DATA_BLOCK "DB_SFB53_FB12"
TITLE =
AUTHOR : SIMATIC
FAMILY : DP
VERSION : 0.1

"WRREC"
BEGIN
   REQ := FALSE;
   ID := DW#16#0;
   INDEX := 0;
   LEN := 0;
   DONE := FALSE;
   BUSY := FALSE;
   ERROR := FALSE;
   STATUS := DW#16#0;
END_DATA_BLOCK

DATA_BLOCK "DB_SFB52_FB10"
TITLE =
AUTHOR : SIMATIC
FAMILY : DP
VERSION : 0.1

"RDREC"
BEGIN
   REQ := FALSE;
   ID := DW#16#0;
   INDEX := 0;
   MLEN := 0;
   VALID := FALSE;
   BUSY := FALSE;
   ERROR := FALSE;
   STATUS := DW#16#0;
   LEN := 0;
END_DATA_BLOCK

DATA_BLOCK "PS_ZYK_DATEN"
TITLE =
VERSION : 0.1
NON_RETAIN


  STRUCT
   Power_Supply : ARRAY  [1 .. 1 ] OF STRUCT
    MESSUNG : STRUCT
     ISTWERT_U : WORD ;
     ISTWERT_I : WORD ;
     ISTWERT_P : WORD ;
    END_STRUCT ;
    PARAMETER : STRUCT
     SCHREIBEN : STRUCT
      SOLLWERT_SPANNUNG : WORD  := W#16#1600;
      SOLLWERT_STROM : WORD  := W#16#A00;
      OPTION_SOLLWERT_LEISTUNG : WORD ;
      OPTION_SOLLWERT_OVP : WORD ;
      OPT_SOLLWERT_WIDERSTAND : WORD ;
     END_STRUCT ;
     LESEN : STRUCT
      STATE : STRUCT
       GERAETEZUSTAND : WORD ;
      END_STRUCT ;
     END_STRUCT ;
    END_STRUCT ;
   END_STRUCT ;
   KONSTANTEN : STRUCT
    LOGISCH_WAHR : BOOL  := TRUE;
    LOGISCH_FALSCH : BOOL ;
   END_STRUCT ;
  END_STRUCT ;
BEGIN
   Power_Supply[1].MESSUNG.ISTWERT_U := W#16#0;
   Power_Supply[1].MESSUNG.ISTWERT_I := W#16#0;
   Power_Supply[1].MESSUNG.ISTWERT_P := W#16#0;
   Power_Supply[1].PARAMETER.SCHREIBEN.SOLLWERT_SPANNUNG := W#16#0;
   Power_Supply[1].PARAMETER.SCHREIBEN.SOLLWERT_STROM := W#16#0;
   Power_Supply[1].PARAMETER.SCHREIBEN.OPTION_SOLLWERT_LEISTUNG := W#16#0;
   Power_Supply[1].PARAMETER.SCHREIBEN.OPTION_SOLLWERT_OVP := W#16#0;
   Power_Supply[1].PARAMETER.SCHREIBEN.OPT_SOLLWERT_WIDERSTAND := W#16#0;
   Power_Supply[1].PARAMETER.LESEN.STATE.GERAETEZUSTAND := W#16#0;
   KONSTANTEN.LOGISCH_WAHR := TRUE;
   KONSTANTEN.LOGISCH_FALSCH := FALSE;
END_DATA_BLOCK

DATA_BLOCK "PS_AZYK_DATEN"
TITLE =
VERSION : 0.1


  STRUCT
   DPV1_Objekte : ARRAY  [1 .. 2 ] OF //vorläufige Platzhaltervariable
   STRUCT
    LESEN : STRUCT
     GERATEDATEN : STRUCT
      GERAETETYP : STRING  [16 ] := 'PSI 9080-100';
      GERAETESERIENNUMMER : STRING  [16 ] := '1026330001';
      GERAETENENNSPANNUNG : REAL  := 8.000000e+001;
      GERAETENENNSTROM : REAL  := 1.000000e+002;
      GERAETEARTIKELNUMMER : STRING  [16 ] := '15200769';
      GERAETEFIRMWARE : STRING  [16 ];
      AKTUELLE_SOLLWERTE : STRUCT
       SPANNUNG : WORD ;
       STROM : WORD ;
       LEISTUNG : WORD ;
      END_STRUCT ;
      GERAETEMELDUNGEN : STRUCT
       KATEGORIE_1 : WORD ;
       CODE_1 : WORD ;
       KATEGORIE_2 : WORD ;
       CODE_2 : WORD ;
       KATEGORIE_3 : WORD ;
       CODE_3 : WORD ;
      END_STRUCT ;
     END_STRUCT ;
    END_STRUCT ;
    SCHREIBEN : STRUCT
     STEUERUNG_GERAET : WORD ;
     SPANNUNGSSOLLWERT : WORD ;
     STROMSOLLWERT : WORD ;
    END_STRUCT ;
   END_STRUCT ;
  END_STRUCT ;
BEGIN
   DPV1_Objekte[1].LESEN.GERATEDATEN.GERAETETYP := 'PSI 9080-100';
   DPV1_Objekte[1].LESEN.GERATEDATEN.GERAETESERIENNUMMER := '';
   DPV1_Objekte[1].LESEN.GERATEDATEN.GERAETENENNSPANNUNG := 0.000000e+000;
   DPV1_Objekte[1].LESEN.GERATEDATEN.GERAETENENNSTROM := 0.000000e+000;
   DPV1_Objekte[1].LESEN.GERATEDATEN.GERAETEARTIKELNUMMER := '';
   DPV1_Objekte[1].LESEN.GERATEDATEN.GERAETEFIRMWARE := '';
   DPV1_Objekte[1].LESEN.GERATEDATEN.AKTUELLE_SOLLWERTE.SPANNUNG := W#16#0;
   DPV1_Objekte[1].LESEN.GERATEDATEN.AKTUELLE_SOLLWERTE.STROM := W#16#0;
   DPV1_Objekte[1].LESEN.GERATEDATEN.AKTUELLE_SOLLWERTE.LEISTUNG := W#16#0;
   DPV1_Objekte[1].LESEN.GERATEDATEN.GERAETEMELDUNGEN.KATEGORIE_1 := W#16#0;
   DPV1_Objekte[1].LESEN.GERATEDATEN.GERAETEMELDUNGEN.CODE_1 := W#16#0;
   DPV1_Objekte[1].LESEN.GERATEDATEN.GERAETEMELDUNGEN.KATEGORIE_2 := W#16#0;
   DPV1_Objekte[1].LESEN.GERATEDATEN.GERAETEMELDUNGEN.CODE_2 := W#16#0;
   DPV1_Objekte[1].LESEN.GERATEDATEN.GERAETEMELDUNGEN.KATEGORIE_3 := W#16#0;
   DPV1_Objekte[1].LESEN.GERATEDATEN.GERAETEMELDUNGEN.CODE_3 := W#16#0;
   DPV1_Objekte[1].SCHREIBEN.STEUERUNG_GERAET := W#16#0;
   DPV1_Objekte[1].SCHREIBEN.SPANNUNGSSOLLWERT := W#16#0;
   DPV1_Objekte[1].SCHREIBEN.STROMSOLLWERT := W#16#0;
   DPV1_Objekte[2].LESEN.GERATEDATEN.GERAETETYP := 'PSI 9080-100';
   DPV1_Objekte[2].LESEN.GERATEDATEN.GERAETESERIENNUMMER := '';
   DPV1_Objekte[2].LESEN.GERATEDATEN.GERAETENENNSPANNUNG := 0.000000e+000;
   DPV1_Objekte[2].LESEN.GERATEDATEN.GERAETENENNSTROM := 0.000000e+000;
   DPV1_Objekte[2].LESEN.GERATEDATEN.GERAETEARTIKELNUMMER := '';
   DPV1_Objekte[2].LESEN.GERATEDATEN.GERAETEFIRMWARE := '';
   DPV1_Objekte[2].LESEN.GERATEDATEN.AKTUELLE_SOLLWERTE.SPANNUNG := W#16#0;
   DPV1_Objekte[2].LESEN.GERATEDATEN.AKTUELLE_SOLLWERTE.STROM := W#16#0;
   DPV1_Objekte[2].LESEN.GERATEDATEN.AKTUELLE_SOLLWERTE.LEISTUNG := W#16#0;
   DPV1_Objekte[2].LESEN.GERATEDATEN.GERAETEMELDUNGEN.KATEGORIE_1 := W#16#0;
   DPV1_Objekte[2].LESEN.GERATEDATEN.GERAETEMELDUNGEN.CODE_1 := W#16#0;
   DPV1_Objekte[2].LESEN.GERATEDATEN.GERAETEMELDUNGEN.KATEGORIE_2 := W#16#0;
   DPV1_Objekte[2].LESEN.GERATEDATEN.GERAETEMELDUNGEN.CODE_2 := W#16#0;
   DPV1_Objekte[2].LESEN.GERATEDATEN.GERAETEMELDUNGEN.KATEGORIE_3 := W#16#0;
   DPV1_Objekte[2].LESEN.GERATEDATEN.GERAETEMELDUNGEN.CODE_3 := W#16#0;
   DPV1_Objekte[2].SCHREIBEN.STEUERUNG_GERAET := W#16#0;
   DPV1_Objekte[2].SCHREIBEN.SPANNUNGSSOLLWERT := W#16#0;
   DPV1_Objekte[2].SCHREIBEN.STROMSOLLWERT := W#16#0;
END_DATA_BLOCK

DATA_BLOCK "WRREC_DB_CONTROLL"
TITLE =
VERSION : 0.1


  STRUCT
   VALID : BOOL ;	//vorläufige Platzhaltervariable
   BUSY : BOOL ;
   ERROR : BOOL ;
   STATUS : DWORD ;
   LAENGE : INT ;
   RECORD : ARRAY  [0 .. 1 ] OF BYTE ;
  END_STRUCT ;
BEGIN
   VALID := FALSE;
   BUSY := FALSE;
   ERROR := FALSE;
   STATUS := DW#16#0;
   LAENGE := 0;
   RECORD[0] := B#16#0;
   RECORD[1] := B#16#0;
END_DATA_BLOCK

DATA_BLOCK "RDREC_DB_DEVICEMESS"
TITLE =
VERSION : 0.1


  STRUCT
   VALID : BOOL ;	//vorläufige Platzhaltervariable
   BUSY : BOOL ;
   ERROR : BOOL ;
   STATUS : DWORD ;
   LAENGE : INT ;
   RECORD : ARRAY  [0 .. 5 ] OF BYTE ;
  END_STRUCT ;
BEGIN
   VALID := FALSE;
   BUSY := FALSE;
   ERROR := FALSE;
   STATUS := DW#16#0;
   LAENGE := 0;
   RECORD[0] := B#16#0;
   RECORD[1] := B#16#0;
   RECORD[2] := B#16#0;
   RECORD[3] := B#16#0;
   RECORD[4] := B#16#0;
   RECORD[5] := B#16#0;
END_DATA_BLOCK

DATA_BLOCK "WRREC_DB_SETVAVOLT"
TITLE =
VERSION : 0.1
NON_RETAIN


  STRUCT
   DONE : BOOL ;	//Datensatz wurde übertragen
   BUSY : BOOL ;	//Schreibvorgang noch nicht beendet (BUSY=1)
   ERROR : BOOL ;	//Schreibvorgang Fehler (ERROR=1)
   STATUS : DWORD ;	//Aufrufkennung / Fehlercode
   RECORD : ARRAY  [0 .. 1 ] OF //Datensatz (zu schreiben)
   BYTE ;
  END_STRUCT ;
BEGIN
   DONE := FALSE;
   BUSY := FALSE;
   ERROR := FALSE;
   STATUS := DW#16#0;
   RECORD[0] := B#16#0;
   RECORD[1] := B#16#0;
END_DATA_BLOCK

DATA_BLOCK "RDREC_DB_ACTSET"
TITLE =
VERSION : 0.1


  STRUCT
   VALID : BOOL ;	//vorläufige Platzhaltervariable
   BUSY : BOOL ;
   ERROR : BOOL ;
   STATUS : DWORD ;
   LAENGE : INT ;
   RECORD : ARRAY  [0 .. 2 ] OF WORD ;
  END_STRUCT ;
BEGIN
   VALID := FALSE;
   BUSY := FALSE;
   ERROR := FALSE;
   STATUS := DW#16#0;
   LAENGE := 0;
   RECORD[0] := W#16#0;
   RECORD[1] := W#16#0;
   RECORD[2] := W#16#0;
END_DATA_BLOCK

DATA_BLOCK "WRREC_DB_SETVACURR"
TITLE =
VERSION : 0.1
NON_RETAIN


  STRUCT
   DONE : BOOL ;	//vorläufige Platzhaltervariable
   BUSY : BOOL ;
   ERROR : BOOL ;
   STATUS : DWORD ;
   RECORD : ARRAY  [0 .. 1 ] OF BYTE ;
  END_STRUCT ;
BEGIN
   DONE := FALSE;
   BUSY := FALSE;
   ERROR := FALSE;
   STATUS := DW#16#0;
   RECORD[0] := B#16#0;
   RECORD[1] := B#16#0;
END_DATA_BLOCK

DATA_BLOCK "RDREC_DB_DEVICETYP"
TITLE =
VERSION : 0.1
NON_RETAIN


  STRUCT
   VALID : BOOL ;	//vorläufige Platzhaltervariable
   BUSY : BOOL ;
   ERROR : BOOL ;
   STATUS : DWORD ;
   LAENGE : INT ;
   RECORD : ARRAY  [0 .. 15 ] OF BYTE ;
  END_STRUCT ;
BEGIN
   VALID := FALSE;
   BUSY := FALSE;
   ERROR := FALSE;
   STATUS := DW#16#0;
   LAENGE := 0;
   RECORD[0] := B#16#0;
   RECORD[1] := B#16#0;
   RECORD[2] := B#16#0;
   RECORD[3] := B#16#0;
   RECORD[4] := B#16#0;
   RECORD[5] := B#16#0;
   RECORD[6] := B#16#0;
   RECORD[7] := B#16#0;
   RECORD[8] := B#16#0;
   RECORD[9] := B#16#0;
   RECORD[10] := B#16#0;
   RECORD[11] := B#16#0;
   RECORD[12] := B#16#0;
   RECORD[13] := B#16#0;
   RECORD[14] := B#16#0;
   RECORD[15] := B#16#0;
END_DATA_BLOCK

DATA_BLOCK "RDREC_DB_DEVARTNO"
TITLE =
VERSION : 0.1
NON_RETAIN


  STRUCT
   VALID : BOOL ;	//vorläufige Platzhaltervariable
   BUSY : BOOL ;
   ERROR : BOOL ;
   STATUS : DWORD ;
   LAENGE : INT ;
   RECORD : ARRAY  [0 .. 15 ] OF BYTE ;
  END_STRUCT ;
BEGIN
   VALID := FALSE;
   BUSY := FALSE;
   ERROR := FALSE;
   STATUS := DW#16#0;
   LAENGE := 0;
   RECORD[0] := B#16#0;
   RECORD[1] := B#16#0;
   RECORD[2] := B#16#0;
   RECORD[3] := B#16#0;
   RECORD[4] := B#16#0;
   RECORD[5] := B#16#0;
   RECORD[6] := B#16#0;
   RECORD[7] := B#16#0;
   RECORD[8] := B#16#0;
   RECORD[9] := B#16#0;
   RECORD[10] := B#16#0;
   RECORD[11] := B#16#0;
   RECORD[12] := B#16#0;
   RECORD[13] := B#16#0;
   RECORD[14] := B#16#0;
   RECORD[15] := B#16#0;
END_DATA_BLOCK

DATA_BLOCK "RDREC_DB_DEVNOMVALUE"
TITLE =
VERSION : 0.1
NON_RETAIN


  STRUCT
   VALID : BOOL ;	//vorläufige Platzhaltervariable
   BUSY : BOOL ;
   ERROR : BOOL ;
   STATUS : DWORD ;
   LAENGE : INT ;
   RECORD : ARRAY  [0 .. 3 ] OF //Nominal Value Voltage
   BYTE ;
  END_STRUCT ;
BEGIN
   VALID := FALSE;
   BUSY := FALSE;
   ERROR := FALSE;
   STATUS := DW#16#0;
   LAENGE := 0;
   RECORD[0] := B#16#0;
   RECORD[1] := B#16#0;
   RECORD[2] := B#16#0;
   RECORD[3] := B#16#0;
END_DATA_BLOCK

DATA_BLOCK "WRREC_DB_SETVAPOW"
TITLE =
VERSION : 0.1


  STRUCT
   DONE : BOOL ;	//vorläufige Platzhaltervariable
   BUSY : BOOL ;
   ERROR : BOOL ;
   STATUS : DWORD ;
   RECORD : ARRAY  [0 .. 1 ] OF BYTE ;
  END_STRUCT ;
BEGIN
   DONE := FALSE;
   BUSY := FALSE;
   ERROR := FALSE;
   STATUS := DW#16#0;
   RECORD[0] := B#16#0;
   RECORD[1] := B#16#0;
END_DATA_BLOCK

DATA_BLOCK "DP_ERROR_DB"
TITLE =
VERSION : 0.1


  STRUCT
   DP_ERROR : BOOL ;	//Slave Fehler
  END_STRUCT ;
BEGIN
   DP_ERROR := FALSE;
END_DATA_BLOCK

FUNCTION "PARA_SPANNUNG_WR" : VOID
TITLE =PARAMETER KONSISTENT SCHREIBEN
VERSION : 0.1


VAR_INPUT
  ADRESSE : INT ;
  DATEN : WORD ;
END_VAR
VAR_TEMP
  _ADRESSE : WORD ;
  _PAFE : INT ;
  _DATEN : WORD ;
END_VAR
BEGIN
NETWORK
TITLE =PARAMETER SPANNUNG SCHREIBEN

      L     #ADRESSE;
      T     #_ADRESSE;

      L     #DATEN;
      T     #_DATEN;

      CALL "DPWR_DAT" (
           LADDR                    := #_ADRESSE,
           RECORD                   := #_DATEN,
           RET_VAL                  := #_PAFE);







END_FUNCTION

FUNCTION "PARA_STROM_WR" : VOID
TITLE =PARAMETER SCHREIBEN
VERSION : 0.1


VAR_INPUT
  ADRESSE : INT ;
  DATEN : WORD ;
END_VAR
VAR_TEMP
  _ADRESSE : WORD ;
  _PAFE : INT ;
  _DATEN : WORD ;
END_VAR
BEGIN
NETWORK
TITLE =PARAMETER STROM SCHREIBEN

      L     #ADRESSE;
      T     #_ADRESSE;

      L     #DATEN;
      T     #_DATEN;

      CALL "DPWR_DAT" (
           LADDR                    := #_ADRESSE,
           RECORD                   := #_DATEN,
           RET_VAL                  := #_PAFE);




END_FUNCTION

FUNCTION "PARA_LEIG_WR" : VOID
TITLE =PARAMETER SCHREIBEN
VERSION : 0.1


VAR_INPUT
  ADRESSE : INT ;
  DATEN : WORD ;
END_VAR
VAR_TEMP
  _ADRESSE : WORD ;
  _PAFE : INT ;
  _DATEN : WORD ;
END_VAR
BEGIN
NETWORK
TITLE =PARAMETER LEISTUNG SCHREIBEN

      L     #ADRESSE;
      T     #_ADRESSE;

      L     #DATEN;
      T     #_DATEN;

      CALL "DPWR_DAT" (
           LADDR                    := #_ADRESSE,
           RECORD                   := P#L 4.0 BYTE 2,
           RET_VAL                  := #_PAFE);

END_FUNCTION

FUNCTION "ISTWERTE_LESEN" : VOID
TITLE =MESSUNG ISTWERTE PS
FAMILY : '        '
NAME : '        '
VERSION : 0.1


VAR_INPUT
  ADRESSE : INT ;
END_VAR
VAR_OUTPUT
  ISTWERT_U : WORD ;
  ISTWERT_I : WORD ;
  ISTWERT_P : WORD ;
END_VAR
VAR_TEMP
  _ADRESSE : WORD ;
  _PAFE : INT ;
  _DATEN : ANY ;
END_VAR
BEGIN
NETWORK
TITLE =ISTWERTE U/I/P LESEN

      L     #ADRESSE;
      T     #_ADRESSE;

      CALL "DPRD_DAT" (
           LADDR                    := #_ADRESSE,
           RET_VAL                  := #_PAFE,
           RECORD                   := P#L 4.0 BYTE 6);//P#DB10.DBX0.0 BYTE 6

      LAR1  P##_DATEN;

      L     LW [AR1,P#0.0];
      T     #ISTWERT_U;

      L     LW [AR1,P#2.0];
      T     #ISTWERT_I;

      L     LW [AR1,P#4.0];
      T     #ISTWERT_P;

END_FUNCTION

FUNCTION "ZUSTAND_LESEN" : VOID
TITLE =GERAETEZUSTAND PS
VERSION : 0.1


VAR_INPUT
  ADRESSE : INT ;
END_VAR
VAR_OUTPUT
  ZUSTAND : WORD ;
END_VAR
VAR_TEMP
  _ADRESSE : WORD ;
  _PAFE : INT ;
  _DATEN : ANY ;
END_VAR
BEGIN
NETWORK
TITLE =GERAETEZUSTAND LESEN

      L     #ADRESSE;
      T     #_ADRESSE;

      CALL "DPRD_DAT" (
           LADDR                    := #_ADRESSE,
           RET_VAL                  := #_PAFE,
           RECORD                   := P#L 4.0 BYTE 2);

      LAR1  P##_DATEN;

      L     LW [AR1,P#0.0];
      T     #ZUSTAND;

END_FUNCTION

FUNCTION "AZYK_WR_SETVALUE" : VOID
TITLE =DPV1 Objekte lesen
VERSION : 0.1


VAR_INPUT
  START : BOOL ;
  ID : DWORD ;
  INDEX : INT ;
  MAX_LAENGE : INT ;
  DBNUMMER : INT ;
END_VAR
VAR_OUTPUT
  DATA_DONE : BOOL ;
  SFB_BUSY : BOOL ;
  SFB_ERROR : BOOL ;
  SFB_STATUS : DWORD ;
END_VAR
VAR_TEMP
  _DBNUMMER : WORD ;
  _MAXLAENGE : INT ;
  _PDATEN : ANY ;
END_VAR
BEGIN
NETWORK
TITLE =

      L     #MAX_LAENGE;
      T     #_MAXLAENGE;

      L     #DBNUMMER;
      T     #_DBNUMMER;

      L     P##_PDATEN;
      LAR1  ;

      L     B#16#10;
      T     B [AR1,P#0.0];

      L     B#16#2;
      T     B [AR1,P#1.0];

      L     #_MAXLAENGE;
      T     W [AR1,P#2.0];

      L     #_DBNUMMER;
      T     W [AR1,P#4.0];

      L     P#DBX 6.0;
      T     D [AR1,P#6.0];

NETWORK
TITLE =

      CALL "WRREC" , "DB_SFB53_FB12" (
           REQ                      := #START,
           ID                       := #ID,
           INDEX                    := #INDEX,
           LEN                      := #_MAXLAENGE,
           DONE                     := #DATA_DONE,
           BUSY                     := #SFB_BUSY,
           ERROR                    := #SFB_ERROR,
           STATUS                   := #SFB_STATUS,
           RECORD                   := #_PDATEN);



END_FUNCTION

FUNCTION "AZYK_WR_CONTROL" : VOID
TITLE =DPV1 Objekte lesen
VERSION : 0.1


VAR_INPUT
  START : BOOL ;
  ID : DWORD ;
  INDEX : INT ;
  MAX_LAENGE : INT ;
  DBNUMMER : INT ;
END_VAR
VAR_OUTPUT
  DATA_DONE : BOOL ;
  SFB_BUSY : BOOL ;
  SFB_ERROR : BOOL ;
  SFB_STATUS : DWORD ;
END_VAR
VAR_TEMP
  _DBNUMMER : WORD ;
  _MAXLAENGE : INT ;
  _PDATEN : ANY ;
END_VAR
BEGIN
NETWORK
TITLE =ANY Zeiger erstellen

      L     #MAX_LAENGE;
      T     #_MAXLAENGE;

      L     #DBNUMMER;
      T     #_DBNUMMER;

      L     P##_PDATEN;
      LAR1  ;

      L     B#16#10;
      T     B [AR1,P#0.0];

      L     B#16#2;
      T     B [AR1,P#1.0];

      L     #_MAXLAENGE;
      T     W [AR1,P#2.0];

      L     #_DBNUMMER;
      T     W [AR1,P#4.0];

      L     P#DBX 8.0;
      T     D [AR1,P#6.0];

NETWORK
TITLE =

      CALL "WRREC" , "DB_SFB53_FB12" (
           REQ                      := #START,
           ID                       := #ID,
           INDEX                    := #INDEX,
           LEN                      := #_MAXLAENGE,
           DONE                     := #DATA_DONE,
           BUSY                     := #SFB_BUSY,
           ERROR                    := #SFB_ERROR,
           STATUS                   := #SFB_STATUS,
           RECORD                   := #_PDATEN);



END_FUNCTION

FUNCTION "AZYK_RD_DEVICEDATA" : VOID
TITLE =
VERSION : 0.1


VAR_INPUT
  START : BOOL ;
  ID : DWORD ;
  INDEX : INT ;
  MAX_LAENGE : INT ;
  DBNUMMER : INT ;
  BITADRESSE : INT ;
  BYTEADRESSE : INT ;
END_VAR
VAR_OUTPUT
  DATA_VALID : BOOL ;
  SFB_BUSY : BOOL ;
  SFB_ERROR : BOOL ;
  SFB_STATUS : DWORD ;
  LAENGE : INT ;
END_VAR
VAR_TEMP
  _DBNUMMER : INT ;
  _MAXLAENGE : INT ;
  _PDATEN : ANY ;
  _BITADRESSE : INT ;
  _BYTEADRESSE : INT ;
END_VAR
BEGIN
NETWORK
TITLE =

      L     #MAX_LAENGE;
      T     #_MAXLAENGE;

      L     #DBNUMMER;
      T     #_DBNUMMER;

      L     #BITADRESSE;
      T     #_BITADRESSE;

      L     #BYTEADRESSE;
      T     #_BYTEADRESSE;

      L     P##_PDATEN;
      LAR1  ;

      L     B#16#10;
      T     B [AR1,P#0.0];

      L     B#16#2;
      T     B [AR1,P#1.0];

      L     #_MAXLAENGE;
      T     W [AR1,P#2.0];

      L     #_DBNUMMER;
      T     W [AR1,P#4.0];

//L     #_BITADRESSE
//UD    DW#16#7
//L     #_BYTEADRESSE
//SLD   3
//OD
//L     B#16#84
//OD
//T     D [AR1,P#6.0]

      L     P#DBX 8.0;
      T     D [AR1,P#6.0];

      CALL "RDREC" , "DB_SFB52_FB10" (
           REQ                      := #START,
           ID                       := #ID,
           INDEX                    := #INDEX,
           MLEN                     := #_MAXLAENGE,
           VALID                    := #DATA_VALID,
           BUSY                     := #SFB_BUSY,
           ERROR                    := #SFB_ERROR,
           STATUS                   := #SFB_STATUS,
           LEN                      := #LAENGE,
           RECORD                   := #_PDATEN);


END_FUNCTION

FUNCTION "AZYK_RD_DEVICENOMVALUE" : VOID
TITLE =
VERSION : 0.1


VAR_INPUT
  START : BOOL ;
  ID : DWORD ;
  INDEX : INT ;
  MAX_LAENGE : INT ;
  DBNUMMER : INT ;
  BITADRESSE : INT ;
  BYTEADRESSE : INT ;
END_VAR
VAR_OUTPUT
  DATA_VALID : BOOL ;
  SFB_BUSY : BOOL ;
  SFB_ERROR : BOOL ;
  SFB_STATUS : DWORD ;
  LAENGE : INT ;
END_VAR
VAR_TEMP
  _DBNUMMER : INT ;
  _MAXLAENGE : INT ;
  _PDATEN : ANY ;
  _BITADRESSE : INT ;
  _BYTEADRESSE : INT ;
END_VAR
BEGIN
NETWORK
TITLE =

      L     #MAX_LAENGE;
      T     #_MAXLAENGE;

      L     #DBNUMMER;
      T     #_DBNUMMER;

      L     #BITADRESSE;
      T     #_BITADRESSE;

      L     #BYTEADRESSE;
      T     #_BYTEADRESSE;

      L     P##_PDATEN;
      LAR1  ;

      L     B#16#10;
      T     B [AR1,P#0.0];

      L     B#16#2;
      T     B [AR1,P#1.0];

      L     #_MAXLAENGE;
      T     W [AR1,P#2.0];

      L     #_DBNUMMER;
      T     W [AR1,P#4.0];

//L     #_BITADRESSE
//UD    DW#16#7
//L     #_BYTEADRESSE
//SLD   3
//OD
//L     B#16#84
//OD
//T     D [AR1,P#6.0]

      L     P#DBX 8.0;
      T     D [AR1,P#6.0];

      CALL "RDREC" , "DB_SFB52_FB10" (
           REQ                      := #START,
           ID                       := #ID,
           INDEX                    := #INDEX,
           MLEN                     := #_MAXLAENGE,
           VALID                    := #DATA_VALID,
           BUSY                     := #SFB_BUSY,
           ERROR                    := #SFB_ERROR,
           STATUS                   := #SFB_STATUS,
           LEN                      := #LAENGE,
           RECORD                   := #_PDATEN);


END_FUNCTION

FUNCTION "AZYK_RD_DATABYTE" : VOID
TITLE =
VERSION : 0.1


VAR_INPUT
  START : BOOL ;
  ID : DWORD ;
  INDEX : INT ;
  MAX_LAENGE : INT ;
  DBNUMMER : INT ;
END_VAR
VAR_OUTPUT
  DATA_VALID : BOOL ;
  SFB_BUSY : BOOL ;
  SFB_ERROR : BOOL ;
  SFB_STATUS : DWORD ;
  LAENGE : INT ;
END_VAR
VAR_TEMP
  _DBNUMMER : INT ;
  _MAXLAENGE : INT ;
  _PDATEN : ANY ;
END_VAR
BEGIN
NETWORK
TITLE =

      L     #MAX_LAENGE;
      T     #_MAXLAENGE;

      L     #DBNUMMER;
      T     #_DBNUMMER;

      L     P##_PDATEN;
      LAR1  ;

      L     B#16#10;
      T     B [AR1,P#0.0];

      L     B#16#2;
      T     B [AR1,P#1.0];

      L     #_MAXLAENGE;
      T     W [AR1,P#2.0];

      L     #_DBNUMMER;
      T     W [AR1,P#4.0];

      L     P#DBX 8.0;
      T     D [AR1,P#6.0];

      CALL "RDREC" , "DB_SFB52_FB10" (
           REQ                      := #START,
           ID                       := #ID,
           INDEX                    := #INDEX,
           MLEN                     := #_MAXLAENGE,
           VALID                    := #DATA_VALID,
           BUSY                     := #SFB_BUSY,
           ERROR                    := #SFB_ERROR,
           STATUS                   := #SFB_STATUS,
           LEN                      := #LAENGE,
           RECORD                   := #_PDATEN);


END_FUNCTION

FUNCTION_BLOCK "PS_ZYKLISCH_DB10"
TITLE =Zyklische Datenverkehr
VERSION : 0.1

BEGIN
NETWORK
TITLE =Messung Istwerte


      CALL "ISTWERTE_LESEN" (
           ADRESSE                  := 256,
           ISTWERT_U                := "PS_ZYK_DATEN".Power_Supply[1].MESSUNG.ISTWERT_U,
           ISTWERT_I                := "PS_ZYK_DATEN".Power_Supply[1].MESSUNG.ISTWERT_I,
           ISTWERT_P                := "PS_ZYK_DATEN".Power_Supply[1].MESSUNG.ISTWERT_P);

NETWORK
TITLE =Geratezustand ermitteln

      CALL "ZUSTAND_LESEN" (
           ADRESSE                  := 262,
           ZUSTAND                  := "PS_ZYK_DATEN".Power_Supply[1].PARAMETER.LESEN.STATE.GERAETEZUSTAND);


END_FUNCTION_BLOCK

FUNCTION "FC10_COPY" : VOID
TITLE =
VERSION : 0.1


VAR_TEMP
  Quelle : ANY ;
  Ziel : ANY ;
END_VAR
BEGIN
NETWORK
TITLE =

      LAR1  P##Quelle;

      L     B#16#10;
      T     LB [AR1,P#0.0];

      L     B#16#2;
      T     LB [AR1,P#1.0];

      L     10;
      T     LW [AR1,P#2.0];

      L     22;
      T     LW [AR1,P#4.0];
      L     P#DBX 11.0;
      T     LD [AR1,P#6.0];

      LAR1  P##Ziel;

      L     B#16#10;
      T     LB [AR1,P#0.0];

      L     B#16#2;
      T     LB [AR1,P#1.0];

      L     10;
      T     LW [AR1,P#2.0];

      L     33;
      T     LW [AR1,P#4.0];
      L     P#DBX 202.0;
      T     LD [AR1,P#6.0];

      CALL "BLKMOV" (
           SRCBLK                   := #Quelle,
           RET_VAL                  := MW    12,
           DSTBLK                   := #Ziel);

END_FUNCTION

FUNCTION_BLOCK "PS_ZYKL_SETVALUE"
TITLE =
VERSION : 0.1

BEGIN
NETWORK
TITLE =Parameter Spannung schreiben


      CALL "PARA_SPANNUNG_WR" (
           ADRESSE                  := 272,
           DATEN                    := "PS_ZYK_DATEN".Power_Supply[1].PARAMETER.SCHREIBEN.SOLLWERT_SPANNUNG);

NETWORK
TITLE =Parameter Strom schreiben


      CALL "PARA_STROM_WR" (
           ADRESSE                  := 274,
           DATEN                    := "PS_ZYK_DATEN".Power_Supply[1].PARAMETER.SCHREIBEN.SOLLWERT_STROM);

NETWORK
TITLE =Parameter Leistung schreiben


      CALL "PARA_LEIG_WR" (
           ADRESSE                  := 276,
           DATEN                    := "PS_ZYK_DATEN".Power_Supply[1].PARAMETER.SCHREIBEN.OPTION_SOLLWERT_LEISTUNG);

END_FUNCTION_BLOCK

FUNCTION_BLOCK "PS_AZYK_SETVAVOLT_WRRD"
TITLE =DPV1 Objekt(e) Sollwert setzen und Aktuelle Sollwerte auslesen
VERSION : 0.1


VAR_OUTPUT
  SFBError : BYTE ;
  SFBStatusOut : DWORD ;
END_VAR
VAR_IN_OUT
  FunctionActivate : BOOL ;	//Anstoßen der Funktion
  FunctionBusy : BOOL ;	//Busybit: Solange TRUE, bis Funktion beendet ist oder TimeOut anspricht
  FunctionDone : BOOL ;	//Zeigt an, daß die Funktion beendet ist (mit oder ohne Fehler)
END_VAR
VAR
  FunctionStaticBusy : BOOL ;	//Speicherbit fuer BusyFlag
  FunctionDPV1WriteDone : BOOL ;
  TimeOutCounter : WORD ;
  SFCRequestLength : INT ;
  FunctionFlag : BOOL ;
END_VAR
VAR_TEMP
  _STATICBusy : BOOL ;
  _SFBError : BOOL ;
  _SFBBusy : BOOL ;
  _SFBDone : BOOL ;
  _SFBValid : BOOL ;
  _SFBStatus : DWORD ;
END_VAR
BEGIN
NETWORK
TITLE =FB Evaluierung

      U     #FunctionActivate;
      FP    #FunctionFlag; // wird weder ein DPV1 Dienst angefragt
      O     #FunctionBusy; // ...noch bearbeitet
      SPBN  END; // so wird der Funktionbaustein beendet
      U     #FunctionStaticBusy; // und wenn zuvor einmal geschrieben wurde
      SPBN  NEWR; // dann NEUE DPV1 ANFRAGE (Request) senden
      U     #FunctionDPV1WriteDone; // Wenn beim DPV1 Dienst WRITE Objekt kein Fehler gemeldet wurde
      SPB   READ; // dann DPV1 Dienst READ Objekt
      SPA   WRIT; // wenn keine READ dann Datensatz schreiben
NEWR: NOP   0; // NEUE DPV1 ANFRAGE (Request)
// Initialisierung
      UN    #FunctionStaticBusy;
      S     #FunctionStaticBusy;
      S     #FunctionBusy;
      R     #FunctionDone;
      L     0;
      T     #SFBError; // Systemfunktionsfehler werden zurueckgesetzt
NETWORK
TITLE =Datensatz Sollwert Spannung setzen

WRIT: NOP   0;
      CALL "AZYK_WR_SETVALUE" (
           START                    := TRUE,
           ID                       := DW#16#108,// PEW276
           INDEX                    := 7,
           MAX_LAENGE               := 2,
           DBNUMMER                 := 153,
           DATA_DONE                := #_SFBDone,
           SFB_BUSY                 := #_SFBBusy,
           SFB_ERROR                := #_SFBError,
           SFB_STATUS               := #_SFBStatus);

// Auswertung der Rueckgabewerte
      U     #_SFBBusy; // wenn die Funktion FC_AZYK_SETVALUE nicht beendet ist,
      SPB   ENDB; // dann Funktionsbaustein Ende
      U     #_SFBError; // wenn Funktion FC_AZYK_SETVALUE keinen Fehler meldet
      SPBN  RD_V; // dann LESEN VORBEREITEN
      SET   ; // Funktion FC_AZYK_SETVALUE hat einen Fehler gemeldet
      R     #FunctionBusy;
      R     #FunctionStaticBusy;
      R     #FunctionDPV1WriteDone;
      S     #FunctionDone;
      L     100; // S7 Fehlercode = 100 laden
      T     #SFBError; // Rueckgabe des Fehlercodes
      L     #_SFBStatus; // Funktionsbaustein Status laden
      T     #SFBStatusOut; // Rückgabe des S7 Fehlercodes
      BEA   ; // Funktionsbaustein wird abgebrochen
// Vorbereiten des des DPV1 Lesedienst
RD_V: NOP   0;
      SET   ;
      S     #FunctionDPV1WriteDone; // nach erfolgreichem WRITEREC Flag setzen

NETWORK
TITLE =Datensatz Aktuelle Sollwerte auslesen

READ: NOP   0;
      CALL "AZYK_RD_DATABYTE" (
           START                    := TRUE,
           ID                       := DW#16#108,// PEW 276
           INDEX                    := 9,
           MAX_LAENGE               := 6,// Anzahl Bytes
           DBNUMMER                 := 154,// Datenbausteinnummer
           DATA_VALID               := #_SFBValid,
           SFB_BUSY                 := #_SFBBusy,
           SFB_ERROR                := #_SFBError,
           SFB_STATUS               := #_SFBStatus,
           LAENGE                   := #SFCRequestLength);

// Auswertung der Rueckgabewerte
      U     #_SFBBusy; // wenn die Funktion FC_AZYKRD_CURRSET nicht beendet ist,
      SPB   ENDB; // dann FunctionBusy Flag setzen
      U     #_SFBError; // wenn bei Datensatz schreiben kein Fehler aufgetreten ist
      SPBN  DATA; // dann Datenauswertung
      L     #TimeOutCounter;
      L     1;
      +I    ;
      T     #TimeOutCounter; // TimeOutCounter += 1
      L     #TimeOutCounter; // Wert von TimeOutCunter laden => AKKU1
      L     300; // Wert 300 laden => AKKU1 => TimeOutCounter => AKKU2
      >=I   ; // VKE = 1 bei AKKU2 >= AKKU1
      SPB   TOUT; // Springe bei VKE = 1 nach TOUT
// wenn der Fehler xx80B5xx gemeldet wird, dann liegt bereits ein anderer DPV1 Auftrag vor
      L     #_SFBStatus;
      UD    DW#16#FFFF00;
      L     DW#16#80B500;
      ==D   ;
// O
//L     #_SFCStatus
//UD    DW#16#FFFF00
//L     DW#16#80B200
//==D
      SPBN  ERR;
      NOP   0;
      SPA   ENDB;
// ein Fehler ist aufgetreten
ERR:  SET   ;
      R     #FunctionBusy;
      R     #FunctionStaticBusy;
      R     #FunctionDPV1WriteDone;
      S     #FunctionDone;
      L     100;
      T     #SFBError;
      L     #_SFBStatus;
      T     #SFBStatusOut;
      L     0;
      T     #TimeOutCounter; // Zeitzähler zurueck setzen
      BEA   ;
DATA: NOP   0;
      S     #FunctionDone;
      R     #FunctionBusy;
      R     #FunctionStaticBusy;
      R     #FunctionDPV1WriteDone;
      R     #FunctionActivate;
      L     0;
      T     #TimeOutCounter;
      BEA   ;

//Timeout
TOUT: NOP   0;
      L     2; // Fehlerwert 2
      T     #SFBError;
      L     0;
      T     #TimeOutCounter; // Zeitzaehler zurueck setzen
      SET   ;
      S     #FunctionDone;
      R     #FunctionActivate;
      R     #FunctionBusy;
      R     #_STATICBusy;
      R     #FunctionDPV1WriteDone;
      BEA   ;
NETWORK
TITLE =Funktionsbaustein definiert beenden

ENDB: SET   ;
      S     #FunctionBusy;
END:  NOP   0;

END_FUNCTION_BLOCK

DATA_BLOCK "DB_FB12_AZYK"
TITLE =
VERSION : 0.1

"PS_AZYK_SETVAVOLT_WRRD"
BEGIN
   SFBError := B#16#0;
   SFBStatusOut := DW#16#0;
   FunctionActivate := FALSE;
   FunctionBusy := FALSE;
   FunctionDone := FALSE;
   FunctionStaticBusy := FALSE;
   FunctionDPV1WriteDone := FALSE;
   TimeOutCounter := W#16#0;
   SFCRequestLength := 0;
   FunctionFlag := FALSE;
END_DATA_BLOCK

FUNCTION_BLOCK "PS_AZYK_SETVACURR_WRRD"
TITLE =DPV1 Objekt(e) Sollwert setzen und Aktuelle Sollwerte auslesen
VERSION : 0.1


VAR_OUTPUT
  SFBError : BYTE ;
  SFBStatusOut : DWORD ;
END_VAR
VAR_IN_OUT
  FunctionActivate : BOOL ;
  FunctionBusy : BOOL ;
  FunctionDone : BOOL ;
END_VAR
VAR
  FunctionStaticBusy : BOOL ;	//SPeicherbit fuer BusyFLag
  FunctionDPV1WriteDone : BOOL ;
  TimeOutCounter : WORD ;
  SFBRequestLength : INT ;
  FunctionFlag : BOOL ;
END_VAR
VAR_TEMP
  _STATICBusy : BOOL ;
  _SFBError : BOOL ;
  _SFBBusy : BOOL ;
  _SFBDone : BOOL ;
  _SFBValid : BOOL ;
  _SFBStatus : DWORD ;
END_VAR
BEGIN
NETWORK
TITLE =FB Evaluierung

      U     #FunctionActivate;
      FP    #FunctionFlag; // wird weder ein DPV1 Dienst angefragt
      O     #FunctionBusy; // ...noch bearbeitet
      SPBN  END; // so wird der Funktionbaustein beendet
      U     #FunctionStaticBusy; // und wenn zuvor einmal geschrieben wurde
      SPBN  NEWR; // dann NEUE DPV1 ANFRAGE (Request) senden
      U     #FunctionDPV1WriteDone; // Wenn beim DPV1 Dienst WRITE Objekt kein Fehler gemeldet wurde
      SPB   READ; // dann DPV1 Dienst READ Objekt
      SPA   WRIT; // wenn keine READ dann Datensatz schreiben
NEWR: NOP   0; // NEUE DPV1 ANFRAGE (Request)
// Initialisierung
      UN    #FunctionStaticBusy;
      S     #FunctionStaticBusy;
      S     #FunctionBusy;
      R     #FunctionDone;
      L     0;
      T     #SFBError; // Systemfunktionsfehler werden zurueckgesetzt

NETWORK
TITLE =Datensatz Sollwert Strom setzen

WRIT: NOP   0;
      CALL "AZYK_WR_SETVALUE" (
           START                    := TRUE,
           ID                       := DW#16#108,
           INDEX                    := 8,
           MAX_LAENGE               := 2,// Anzahl Bytes
           DBNUMMER                 := 155,// Datenbausteinnummer
           DATA_DONE                := #_SFBDone,
           SFB_BUSY                 := #_SFBBusy,
           SFB_ERROR                := #_SFBError,
           SFB_STATUS               := #_SFBStatus);

// Auswertung der Rueckgabewerte
      U     #_SFBBusy; // wenn die Funktion FC_AZYK_SETVALUE nicht beendet ist,
      SPB   ENDB; // dann Funktionsbaustein Ende
      U     #_SFBError; // wenn Funktion FC_AZYK_SETVALUE keinen Fehler meldet
      SPBN  RD_V; // dann LESEN VORBEREITEN
      SET   ; // Funktion FC_AZYK_SETVALUE hat einen Fehler gemeldet
      R     #FunctionBusy;
      R     #FunctionStaticBusy;
      R     #FunctionDPV1WriteDone;
      S     #FunctionDone;
      L     100; // S7 Fehlercode = 100 laden
      T     #SFBError; // Rueckgabe des Fehlercodes
      L     #_SFBStatus; // Funktionsbaustein Status laden
      T     #SFBStatusOut; // Rückgabe des S7 Fehlercodes
      BEA   ; // Funktionsbaustein wird abgebrochen
// Vorbereiten des DPV1 Lesedienst
RD_V: NOP   0;
      SET   ;
      S     #FunctionDPV1WriteDone; // nach erfolgreichem WRITEREC Flag setzen

NETWORK
TITLE =Datensatz Aktuelle Sollwerte auslesen

READ: NOP   0;
      CALL "AZYK_RD_DATABYTE" (
           START                    := TRUE,
           ID                       := DW#16#108,
           INDEX                    := 9,
           MAX_LAENGE               := 6,// Anzahl Bytes
           DBNUMMER                 := 154,// Datenbausteinnummer
           DATA_VALID               := #_SFBValid,
           SFB_BUSY                 := #_SFBBusy,
           SFB_ERROR                := #_SFBError,
           SFB_STATUS               := #_SFBStatus,
           LAENGE                   := #SFBRequestLength);

// Auswertung der Rueckgabewerte
      U     #_SFBBusy; // wenn die Funktion FC_AZYKRD_CURRSET nicht beendet ist,
      SPB   ENDB; // dann FunctionBusy Flag setzen
      U     #_SFBError; // wenn bei Datensatz schreiben kein Fehler aufgetreten ist
      SPBN  DATA; // dann Datenauswertung
      L     #TimeOutCounter;
      L     1;
      +I    ;
      T     #TimeOutCounter; // TimeOutCounter += 1
      L     #TimeOutCounter; // Wert von TimeOutCunter laden => AKKU1
      L     300; // Wert 300 laden => AKKU1 => TimeOutCounter => AKKU2
      >=I   ; // VKE = 1 bei AKKU2 >= AKKU1
      SPB   TOUT; // Springe bei VKE = 1 nach TOUT
// wenn der Fehler xx80B5xx gemeldet wird, dann liegt bereits ein anderer DPV1 Auftrag vor
      L     #_SFBStatus;
      UD    DW#16#FFFF00;
      L     DW#16#80B500;
      ==D   ;
// O
//L     #_SFCStatus
//UD    DW#16#FFFF00
//L     DW#16#80B200
//==D
      SPBN  ERR;
      NOP   0;
      SPA   ENDB;
// ein Fehler ist aufgetreten
ERR:  SET   ;
      R     #FunctionBusy;
      R     #FunctionStaticBusy;
      R     #FunctionDPV1WriteDone;
      S     #FunctionDone;
      L     100;
      T     #SFBError;
      L     #_SFBStatus;
      T     #SFBStatusOut;
      L     0;
      T     #TimeOutCounter; // Zeitzähler zurueck setzen
      BEA   ;
DATA: NOP   0;
      S     #FunctionDone;
      R     #FunctionBusy;
      R     #FunctionStaticBusy;
      R     #FunctionDPV1WriteDone;
      R     #FunctionActivate;
      L     0;
      T     #TimeOutCounter;
      BEA   ;

//Timeout
TOUT: NOP   0;
      L     2; // Fehlerwert 2
      T     #SFBError;
      L     0;
      T     #TimeOutCounter; // Zeitzaehler zurueck setzen
      SET   ;
      S     #FunctionDone;
      R     #FunctionActivate;
      R     #FunctionBusy;
      R     #_STATICBusy;
      R     #FunctionDPV1WriteDone;
      BEA   ;
NETWORK
TITLE =Funktionsbaustein definiert beenden

ENDB: SET   ;
      S     #FunctionBusy;
END:  NOP   0;

END_FUNCTION_BLOCK

DATA_BLOCK "DB_FB13_AZYK"
TITLE =
VERSION : 0.0

"PS_AZYK_SETVACURR_WRRD"
BEGIN
   SFBError := B#16#0;
   SFBStatusOut := DW#16#0;
   FunctionActivate := FALSE;
   FunctionBusy := FALSE;
   FunctionDone := FALSE;
   FunctionStaticBusy := FALSE;
   FunctionDPV1WriteDone := FALSE;
   TimeOutCounter := W#16#0;
   SFBRequestLength := 0;
   FunctionFlag := FALSE;
END_DATA_BLOCK

FUNCTION_BLOCK "PS_AZYK_CONTROLL_WRRD"
TITLE =DPV1 Objekt Geraet Steuerung
VERSION : 0.1


VAR_INPUT
  DBNummer_STEUERN : INT ;
  Datensatznr_STEUERN : INT ;
  DBNummer_MELDUNGEN : INT ;
  Datensatznr_MELDUNGEN : INT ;
END_VAR
VAR_OUTPUT
  SFBError : BYTE ;
  SFBStatusOut : DWORD ;
END_VAR
VAR_IN_OUT
  FunctionActivate : BOOL ;
  FunctionBusy : BOOL ;
  FunctionDone : BOOL ;
END_VAR
VAR
  FunctionStaticBusy : BOOL ;	//SPeicherbit fuer BusyFLag
  FunctionDPV1WriteDone : BOOL ;
  TimeOutCounter : WORD ;
  SFBRequestLength : INT ;
  FunctionFlag : BOOL ;
END_VAR
VAR_TEMP
  _STATICBusy : BOOL ;
  _SFBError : BOOL ;
  _SFBBusy : BOOL ;
  _SFBDone : BOOL ;
  _SFBValid : BOOL ;
  _SFBStatus : DWORD ;
END_VAR
BEGIN
NETWORK
TITLE =FB Evaluierung

      U     #FunctionActivate;
      FP    #FunctionFlag; // wird weder ein DPV1 Dienst angefragt
      O     #FunctionBusy; // ...noch bearbeitet
      SPBN  END; // so wird der Funktionbaustein beendet
      U     #FunctionStaticBusy; // und wenn zuvor einmal geschrieben wurde
      SPBN  NEWR; // dann NEUE DPV1 ANFRAGE (Request) senden
      U     #FunctionDPV1WriteDone; // Wenn beim DPV1 Dienst WRITE Objekt kein Fehler gemeldet wurde
      SPB   READ; // dann DPV1 Dienst READ Objekt
      SPA   WRIT; // wenn keine READ dann Datensatz schreiben
NEWR: NOP   0; // NEUE DPV1 ANFRAGE (Request)
// Initialisierung
      UN    #FunctionStaticBusy;
      S     #FunctionStaticBusy;
      S     #FunctionBusy;
      R     #FunctionDone;
      L     0;
      T     #SFBError; // Systemfunktionsfehler werden zurueckgesetzt

NETWORK
TITLE =Datensatz Geraet steuern

WRIT: NOP   0;
      CALL "AZYK_WR_CONTROL" (
           START                    := TRUE,
           ID                       := DW#16#108,
           INDEX                    := #Datensatznr_STEUERN,
           MAX_LAENGE               := 2,
           DBNUMMER                 := #DBNummer_STEUERN,
           DATA_DONE                := #_SFBDone,
           SFB_BUSY                 := #_SFBBusy,
           SFB_ERROR                := #_SFBError,
           SFB_STATUS               := #_SFBStatus);


// Auswertung der Rueckgabewerte
      U     #_SFBBusy; // wenn die Funktion FC_AZYK_SETVALUE nicht beendet ist,
      SPB   ENDB; // dann Funktionsbaustein Ende
      U     #_SFBError; // wenn Funktion FC_AZYK_SETVALUE keinen Fehler meldet
      SPBN  RD_V; // dann LESEN VORBEREITEN
      SET   ; // Funktion FC_AZYK_SETVALUE hat einen Fehler gemeldet
      R     #FunctionBusy;
      R     #FunctionStaticBusy;
      R     #FunctionDPV1WriteDone;
      S     #FunctionDone;
      L     100; // Fehlercode = 100 laden
      T     #SFBError; // Rueckgabe des Fehlercodes
      L     #_SFBStatus; // Funktionsbaustein Status laden
      T     #SFBStatusOut; // Rückgabe des Statuswert
      BEA   ; // Funktionsbaustein wird abgebrochen
// Vorbereiten des des DPV1 Lesedienst
RD_V: NOP   0;
      SET   ;
      S     #FunctionDPV1WriteDone; // nach erfolgreichem WRITEREC Flag setzen

NETWORK
TITLE =Datensatz Geraetemeldungen auslesen

READ: NOP   0;
      CALL "AZYK_RD_DATABYTE" (
           START                    := TRUE,
           ID                       := DW#16#108,
           INDEX                    := #Datensatznr_MELDUNGEN,
           MAX_LAENGE               := 6,// Anzahl in Bytes
           DBNUMMER                 := #DBNummer_MELDUNGEN,// Datenbausteinnummer
           DATA_VALID               := #_SFBValid,
           SFB_BUSY                 := #_SFBBusy,
           SFB_ERROR                := #_SFBError,
           SFB_STATUS               := #_SFBStatus,
           LAENGE                   := #SFBRequestLength);

// Auswertung der Rueckgabewerte
      U     #_SFBBusy; // wenn die Funktion FC_AZYKRD_CURRSET nicht beendet ist,
      SPB   ENDB; // dann FunctionBusy Flag setzen
      U     #_SFBError; // wenn bei Datensatz schreiben kein Fehler aufgetreten ist
      SPBN  DATA; // dann Datenauswertung
      L     #TimeOutCounter;
      L     1;
      +I    ;
      T     #TimeOutCounter; // TimeOutCounter += 1
      L     #TimeOutCounter; // Wert von TimeOutCunter laden => AKKU1
      L     300; // Wert 300 laden => AKKU1 => TimeOutCounter => AKKU2
      >=I   ; // VKE = 1 bei AKKU2 >= AKKU1
      SPB   TOUT; // Springe bei VKE = 1 nach TOUT
// wenn der Fehler xx80B5xx gemeldet wird, dann liegt bereits ein anderer DPV1 Auftrag vor
      L     #_SFBStatus;
      UD    DW#16#FFFF00;
      L     DW#16#80B500;
      ==D   ;
      O     ;
// wenn der Fehler xx80B2xx gemeldet wird, ist die vorliegende Projektierung der Steckplatzdefinition fehlerhaft
//      L     #_SFBStatus
//      UD    DW#16#FFFF00
//      L     DW#16#80B200
//      ==D
      SPBN  ERR;
      NOP   0;
      SPA   ENDB;
// ein Fehler ist aufgetreten
ERR:  SET   ;
      R     #FunctionBusy;
      R     #FunctionStaticBusy;
      R     #FunctionDPV1WriteDone;
      S     #FunctionDone;
      L     100;
      T     #SFBError;
      L     #_SFBStatus;
      T     #SFBStatusOut;
      L     0;
      T     #TimeOutCounter; // Zeitzähler zurueck setzen
      BEA   ;
DATA: NOP   0;
      S     #FunctionDone;
      R     #FunctionBusy;
      R     #FunctionStaticBusy;
      R     #FunctionDPV1WriteDone;
      R     #FunctionActivate;
      L     0;
      T     #TimeOutCounter; // Zeitzähler zurück setzen
      BEA   ;

//Timeout
TOUT: NOP   0;
      L     2; // Fehlerwert 2
      T     #SFBError;
      L     0;
      T     #TimeOutCounter; // Zeitzaehler zurueck setzen
      SET   ;
      S     #FunctionDone;
      R     #FunctionActivate;
      R     #FunctionBusy;
      R     #_STATICBusy;
      R     #FunctionDPV1WriteDone;
      BEA   ;
NETWORK
TITLE =Funktionsbaustein definiert beenden

ENDB: SET   ;
      S     #FunctionBusy;
END:  NOP   0;

END_FUNCTION_BLOCK

DATA_BLOCK "DB_FB14_AZYK"
TITLE =
VERSION : 0.0

"PS_AZYK_CONTROLL_WRRD"
BEGIN
   DBNummer_STEUERN := 0;
   Datensatznr_STEUERN := 0;
   DBNummer_MELDUNGEN := 0;
   Datensatznr_MELDUNGEN := 0;
   SFBError := B#16#0;
   SFBStatusOut := DW#16#0;
   FunctionActivate := FALSE;
   FunctionBusy := FALSE;
   FunctionDone := FALSE;
   FunctionStaticBusy := FALSE;
   FunctionDPV1WriteDone := FALSE;
   TimeOutCounter := W#16#0;
   SFBRequestLength := 0;
   FunctionFlag := FALSE;
END_DATA_BLOCK

FUNCTION_BLOCK "PS_AZYK_DEVICETYP_RD"
TITLE =DPV1 Objekt Geraetetyp
VERSION : 0.1


VAR_INPUT
  DBNummer_DEVICETYP : INT ;
  Datensatznr_DEVICETYP : INT ;
END_VAR
VAR_OUTPUT
  SFBError : BYTE ;
  SFBStatusOut : DWORD ;
END_VAR
VAR_IN_OUT
  FunctionActivate : BOOL ;
  FunctionBusy : BOOL ;
  FunctionDone : BOOL ;
END_VAR
VAR
  FunctionStaticBusy : BOOL ;	//SPeicherbit fuer BusyFLag
  FunctionDPV1WriteDone : BOOL ;
  TimeOutCounter : WORD ;
  SFBRequestLength : INT ;
  FunctionFlag : BOOL ;
END_VAR
VAR_TEMP
  _STATICBusy : BOOL ;
  _SFBError : BOOL ;
  _SFBBusy : BOOL ;
  _SFBDone : BOOL ;
  _SFBValid : BOOL ;
  _SFBStatus : DWORD ;
END_VAR
BEGIN
NETWORK
TITLE =FB Evaluierung

      U     #FunctionActivate;
      FP    #FunctionFlag;
      O     #FunctionBusy; // Sollwert wird noch gesetzt
      SPBN  END; // Funktionbaustein wird beendet wenn nicht..
      U     #FunctionStaticBusy; // und wenn zuvor einmal geschrieben wurde
      SPBN  NEWR; // dann NEUE DPV1 ANFRAGE ansonsten
      SPA   READ;
NEWR: NOP   0; // NEUE DPV1 ANFRAGE
// Initialisierung
      UN    #FunctionStaticBusy;
      S     #FunctionStaticBusy;
      S     #FunctionBusy;
      R     #FunctionDone;
      L     0;
      T     #SFBError; // Systemfunktionsfehler werden zurueckgesetzt
NETWORK
TITLE =Datensatz Geraetetyp lesen

READ: NOP   0;

      CALL "AZYK_RD_DEVICEDATA" (
           START                    := TRUE,
           ID                       := DW#16#108,
           INDEX                    := #Datensatznr_DEVICETYP,
           MAX_LAENGE               := 16,
           DBNUMMER                 := #DBNummer_DEVICETYP,
           BITADRESSE               := 0,
           BYTEADRESSE              := 8,
           DATA_VALID               := #_SFBValid,
           SFB_BUSY                 := #_SFBBusy,
           SFB_ERROR                := #_SFBError,
           SFB_STATUS               := #_SFBStatus,
           LAENGE                   := #SFBRequestLength);

// Auswertung der Rueckgabewerte
      U     #_SFBBusy; // wenn die Funktion FC_AZYKRD_CURRSET nicht beendet ist,
      SPB   ENDB; // dann FunctionBusy Flag setzen
      U     #_SFBError; // wenn bei Datensatz schreiben kein Fehler aufgetreten ist
      SPBN  DATA; // dann Datenauswertung
      L     #TimeOutCounter;
      L     1;
      +I    ;
      T     #TimeOutCounter; // TimeOutCounter += 1
      L     #TimeOutCounter; // Wert von TimeOutCunter laden => AKKU1
      L     300; // Wert 300 laden => AKKU1 => TimeOutCounter => AKKU2
      >=I   ; // VKE = 1 bei AKKU2 >= AKKU1
      SPB   TOUT; // Springe bei VKE = 1 nach TOUT
// wenn der Fehler xx80B5xx gemeldet wird, dann liegt bereits ein anderer DPV1 Auftrag vor
      L     #_SFBStatus;
      UD    DW#16#FFFF00;
      L     DW#16#80B500;
      ==D   ;
      SPBN  ERR;
      NOP   0;
      SPA   ENDB;
// ein Fehler ist aufgetreten
ERR:  SET   ;
      R     #FunctionBusy;
      R     #FunctionStaticBusy;
      R     #FunctionDPV1WriteDone;
      S     #FunctionDone;
      L     100;
      T     #SFBError;
      L     #_SFBStatus;
      T     #SFBStatusOut;
      L     0;
      T     #TimeOutCounter; // Zeitzähler zurueck setzen
      BEA   ;
DATA: NOP   0;
      S     #FunctionDone;
      R     #FunctionBusy;
      R     #FunctionStaticBusy;
      R     #FunctionDPV1WriteDone;
      R     #FunctionActivate;
      L     0;
      T     #TimeOutCounter; // Zeitzähler zurück setzen
      BEA   ;

//Timeout
TOUT: NOP   0;
      L     2; // Fehlerwert 2
      T     #SFBError;
      L     0;
      T     #TimeOutCounter; // Zeitzaehler zurueck setzen
      SET   ;
      S     #FunctionDone;
      R     #FunctionActivate;
      R     #FunctionBusy;
      R     #_STATICBusy;
      R     #FunctionDPV1WriteDone;
      BEA   ;
NETWORK
TITLE =Funktionsbaustein definiert beenden

ENDB: SET   ;
      S     #FunctionBusy;
END:  NOP   0;

END_FUNCTION_BLOCK

DATA_BLOCK "DB_FB15_AZYK"
TITLE =
VERSION : 0.0

"PS_AZYK_DEVICETYP_RD"
BEGIN
   DBNummer_DEVICETYP := 0;
   Datensatznr_DEVICETYP := 0;
   SFBError := B#16#0;
   SFBStatusOut := DW#16#0;
   FunctionActivate := FALSE;
   FunctionBusy := FALSE;
   FunctionDone := FALSE;
   FunctionStaticBusy := FALSE;
   FunctionDPV1WriteDone := FALSE;
   TimeOutCounter := W#16#0;
   SFBRequestLength := 0;
   FunctionFlag := FALSE;
END_DATA_BLOCK

FUNCTION_BLOCK "PS_AZYK_DEVICEARTNO"
TITLE =DPV1 Objekt Artikelnummer lesen
VERSION : 0.1


VAR_INPUT
  DBNummer_DEVICEARTNO : INT ;
  Datensatznr_DEVICEARTNO : INT ;
END_VAR
VAR_OUTPUT
  SFBError : BYTE ;
  SFBStatusOut : DWORD ;
END_VAR
VAR_IN_OUT
  FunctionActivate : BOOL ;
  FunctionBusy : BOOL ;
  FunctionDone : BOOL ;
END_VAR
VAR
  FunctionStaticBusy : BOOL ;	//SPeicherbit fuer BusyFLag
  FunctionDPV1WriteDone : BOOL ;
  TimeOutCounter : WORD ;
  SFBRequestLength : INT ;
  FunctionFlag : BOOL ;
END_VAR
VAR_TEMP
  _STATICBusy : BOOL ;
  _SFBError : BOOL ;
  _SFBBusy : BOOL ;
  _SFBDone : BOOL ;
  _SFBValid : BOOL ;
  _SFBStatus : DWORD ;
END_VAR
BEGIN
NETWORK
TITLE =FB Evaluierung

      U     #FunctionActivate;
      FP    #FunctionFlag;
      O     #FunctionBusy; // Sollwert wird noch gesetzt
      SPBN  END; // Funktionbaustein wird beendet wenn nicht..
      U     #FunctionStaticBusy; // und wenn zuvor einmal geschrieben wurde
      SPBN  NEWR; // dann NEUE DPV1 ANFRAGE ansonsten
      SPA   READ;
NEWR: NOP   0; // NEUE DPV1 ANFRAGE
// Initialisierung
      UN    #FunctionStaticBusy;
      S     #FunctionStaticBusy;
      S     #FunctionBusy;
      R     #FunctionDone;
      L     0;
      T     #SFBError; // Systemfunktionsfehler werden zurueckgesetzt
NETWORK
TITLE =Datensatz Artikelnummer lesen

READ: NOP   0;

      CALL "AZYK_RD_DEVICEDATA" (
           START                    := TRUE,
           ID                       := DW#16#108,
           INDEX                    := #Datensatznr_DEVICEARTNO,
           MAX_LAENGE               := 16,
           DBNUMMER                 := #DBNummer_DEVICEARTNO,
           BITADRESSE               := 0,
           BYTEADRESSE              := 8,
           DATA_VALID               := #_SFBValid,
           SFB_BUSY                 := #_SFBBusy,
           SFB_ERROR                := #_SFBError,
           SFB_STATUS               := #_SFBStatus,
           LAENGE                   := #SFBRequestLength);

// Auswertung der Rueckgabewerte
      U     #_SFBBusy; // wenn die Funktion FC_AZYKRD_CURRSET nicht beendet ist,
      SPB   ENDB; // dann FunctionBusy Flag setzen
      U     #_SFBError; // wenn bei Datensatz schreiben kein Fehler aufgetreten ist
      SPBN  DATA; // dann Datenauswertung
      L     #TimeOutCounter;
      L     1;
      +I    ;
      T     #TimeOutCounter; // TimeOutCounter += 1
      L     #TimeOutCounter; // Wert von TimeOutCunter laden => AKKU1
      L     300; // Wert 300 laden => AKKU1 => TimeOutCounter => AKKU2
      >=I   ; // VKE = 1 bei AKKU2 >= AKKU1
      SPB   TOUT; // Springe bei VKE = 1 nach TOUT
// wenn der Fehler xx80B5xx gemeldet wird, dann liegt bereits ein anderer DPV1 Auftrag vor
      L     #_SFBStatus;
      UD    DW#16#FFFF00;
      L     DW#16#80B500;
      ==D   ;
      SPBN  ERR;
      NOP   0;
      SPA   ENDB;
// ein Fehler ist aufgetreten
ERR:  SET   ;
      R     #FunctionBusy;
      R     #FunctionStaticBusy;
      R     #FunctionDPV1WriteDone;
      S     #FunctionDone;
      L     100;
      T     #SFBError;
      L     #_SFBStatus;
      T     #SFBStatusOut;
      L     0;
      T     #TimeOutCounter; // Zeitzähler zurueck setzen
      BEA   ;
DATA: NOP   0;
      S     #FunctionDone;
      R     #FunctionBusy;
      R     #FunctionStaticBusy;
      R     #FunctionDPV1WriteDone;
      R     #FunctionActivate;
      L     0;
      T     #TimeOutCounter; // Zeitzähler zurück setzen
      BEA   ;

//Timeout
TOUT: NOP   0;
      L     2; // Fehlerwert 2
      T     #SFBError;
      L     0;
      T     #TimeOutCounter; // Zeitzaehler zurueck setzen
      SET   ;
      S     #FunctionDone;
      R     #FunctionActivate;
      R     #FunctionBusy;
      R     #_STATICBusy;
      R     #FunctionDPV1WriteDone;
      BEA   ;
NETWORK
TITLE =Funktionsbaustein definiert beenden

ENDB: SET   ;
      S     #FunctionBusy;
END:  NOP   0;

END_FUNCTION_BLOCK

DATA_BLOCK "DB_FB16_AZYK"
TITLE =
VERSION : 0.1

"PS_AZYK_DEVICEARTNO"
BEGIN
   DBNummer_DEVICEARTNO := 0;
   Datensatznr_DEVICEARTNO := 0;
   SFBError := B#16#0;
   SFBStatusOut := DW#16#0;
   FunctionActivate := FALSE;
   FunctionBusy := FALSE;
   FunctionDone := FALSE;
   FunctionStaticBusy := FALSE;
   FunctionDPV1WriteDone := FALSE;
   TimeOutCounter := W#16#0;
   SFBRequestLength := 0;
   FunctionFlag := FALSE;
END_DATA_BLOCK

FUNCTION_BLOCK "PS_AZYK_DEVICENOMVALUE"
TITLE =DPV1 Objekt Nennwert Spannung lesen
VERSION : 0.1


VAR_INPUT
  DBNummer_DEVICENOMVALUE : INT ;
  Datensatznr_DEVICENOMVAL : INT ;
END_VAR
VAR_OUTPUT
  SFBError : BYTE ;
  SFBStatusOut : DWORD ;
END_VAR
VAR_IN_OUT
  FunctionActivate : BOOL ;
  FunctionBusy : BOOL ;
  FunctionDone : BOOL ;
END_VAR
VAR
  FunctionStaticBusy : BOOL ;	//SPeicherbit fuer BusyFLag
  FunctionDPV1WriteDone : BOOL ;
  TimeOutCounter : WORD ;
  SFBRequestLength : INT ;
  FunctionFlag : BOOL ;
END_VAR
VAR_TEMP
  _STATICBusy : BOOL ;
  _SFBError : BOOL ;
  _SFBBusy : BOOL ;
  _SFBDone : BOOL ;
  _SFBValid : BOOL ;
  _SFBStatus : DWORD ;
END_VAR
BEGIN
NETWORK
TITLE =FB Evaluierung

      U     #FunctionActivate;
      FP    #FunctionFlag;
      O     #FunctionBusy; // Sollwert wird noch gesetzt
      SPBN  END; // Funktionbaustein wird beendet wenn nicht..
      U     #FunctionStaticBusy; // und wenn zuvor einmal geschrieben wurde
      SPBN  NEWR; // dann NEUE DPV1 ANFRAGE ansonsten
      SPA   READ;
NEWR: NOP   0; // NEUE DPV1 ANFRAGE
// Initialisierung
      UN    #FunctionStaticBusy;
      S     #FunctionStaticBusy;
      S     #FunctionBusy;
      R     #FunctionDone;
      L     0;
      T     #SFBError; // Systemfunktionsfehler werden zurueckgesetzt
NETWORK
TITLE =Datensatz Nennwert Spannung lesen

READ: NOP   0;

      CALL "AZYK_RD_DEVICENOMVALUE" (
           START                    := TRUE,
           ID                       := DW#16#108,
           INDEX                    := #Datensatznr_DEVICENOMVAL,
           MAX_LAENGE               := 4,
           DBNUMMER                 := #DBNummer_DEVICENOMVALUE,
           BITADRESSE               := 0,
           BYTEADRESSE              := 8,
           DATA_VALID               := #_SFBValid,
           SFB_BUSY                 := #_SFBBusy,
           SFB_ERROR                := #_SFBError,
           SFB_STATUS               := #_SFBStatus,
           LAENGE                   := #SFBRequestLength);

// Auswertung der Rueckgabewerte
      U     #_SFBBusy; // wenn die Funktion FC_AZYKRD_CURRSET nicht beendet ist,
      SPB   ENDB; // dann FunctionBusy Flag setzen
      U     #_SFBError; // wenn bei Datensatz schreiben kein Fehler aufgetreten ist
      SPBN  DATA; // dann Datenauswertung
      L     #TimeOutCounter;
      L     1;
      +I    ;
      T     #TimeOutCounter; // TimeOutCounter += 1
      L     #TimeOutCounter; // Wert von TimeOutCunter laden => AKKU1
      L     300; // Wert 300 laden => AKKU1 => TimeOutCounter => AKKU2
      >=I   ; // VKE = 1 bei AKKU2 >= AKKU1
      SPB   TOUT; // Springe bei VKE = 1 nach TOUT
// wenn der Fehler xx80B5xx gemeldet wird, dann liegt bereits ein anderer DPV1 Auftrag vor
      L     #_SFBStatus;
      UD    DW#16#FFFF00;
      L     DW#16#80B500;
      ==D   ;
      SPBN  ERR;
      NOP   0;
      SPA   ENDB;
// ein Fehler ist aufgetreten
ERR:  SET   ;
      R     #FunctionBusy;
      R     #FunctionStaticBusy;
      R     #FunctionDPV1WriteDone;
      S     #FunctionDone;
      L     100;
      T     #SFBError;
      L     #_SFBStatus;
      T     #SFBStatusOut;
      L     0;
      T     #TimeOutCounter; // Zeitzähler zurueck setzen
      BEA   ;
DATA: NOP   0;
      S     #FunctionDone;
      R     #FunctionBusy;
      R     #FunctionStaticBusy;
      R     #FunctionDPV1WriteDone;
      R     #FunctionActivate;
      L     0;
      T     #TimeOutCounter; // Zeitzähler zurück setzen
      BEA   ;

//Timeout
TOUT: NOP   0;
      L     2; // Fehlerwert 2
      T     #SFBError;
      L     0;
      T     #TimeOutCounter; // Zeitzaehler zurueck setzen
      SET   ;
      S     #FunctionDone;
      R     #FunctionActivate;
      R     #FunctionBusy;
      R     #_STATICBusy;
      R     #FunctionDPV1WriteDone;
      BEA   ;
NETWORK
TITLE =Funktionsbaustein definiert beenden

ENDB: SET   ;
      S     #FunctionBusy;
END:  NOP   0;

END_FUNCTION_BLOCK

DATA_BLOCK "DB_FB17_AZYK"
TITLE =
VERSION : 0.0

"PS_AZYK_DEVICENOMVALUE"
BEGIN
   DBNummer_DEVICENOMVALUE := 0;
   Datensatznr_DEVICENOMVAL := 0;
   SFBError := B#16#0;
   SFBStatusOut := DW#16#0;
   FunctionActivate := FALSE;
   FunctionBusy := FALSE;
   FunctionDone := FALSE;
   FunctionStaticBusy := FALSE;
   FunctionDPV1WriteDone := FALSE;
   TimeOutCounter := W#16#0;
   SFBRequestLength := 0;
   FunctionFlag := FALSE;
END_DATA_BLOCK

FUNCTION_BLOCK "PS_AZYK_SETVAPOW_WRRD"
TITLE =DPV1 Objekt(e) Sollwert setzen und aktuelle Solllwerte auslesen
VERSION : 0.1


VAR_OUTPUT
  SFBError : BYTE ;
  SFBStatusOut : DWORD ;
END_VAR
VAR_IN_OUT
  FunctionActivate : BOOL ;
  FunctionBusy : BOOL ;
  FunctionDone : BOOL ;
END_VAR
VAR
  FunctionStaticBusy : BOOL ;
  FunctionDPV1WriteDone : BOOL ;
  TimeOutCounter : WORD ;
  SFBRequestLength : INT ;
  FunctionFlag : BOOL ;
END_VAR
VAR_TEMP
  _STATICBusy : BOOL ;
  _SFBError : BOOL ;
  _SFBBusy : BOOL ;
  _SFBDone : BOOL ;
  _SFBValid : BOOL ;
  _SFBStatus : DWORD ;
END_VAR
BEGIN
NETWORK
TITLE =FB Evaluierung

      U     #FunctionActivate;
      FP    #FunctionFlag; // wird weder ein DPV1 Dienst angefragt
      O     #FunctionBusy; // ...noch bearbeitet
      SPBN  END; // so wird der Funktionbaustein beendet
      U     #FunctionStaticBusy; // und wenn zuvor einmal geschrieben wurde
      SPBN  NEWR; // dann NEUE DPV1 ANFRAGE (Request) senden
      U     #FunctionDPV1WriteDone; // Wenn beim DPV1 Dienst WRITE Objekt kein Fehler gemeldet wurde
      SPB   READ; // dann DPV1 Dienst READ Objekt
      SPA   WRIT; // wenn keine READ dann Datensatz schreiben
NEWR: NOP   0; // NEUE DPV1 ANFRAGE (Request)
// Initialisierung
      UN    #FunctionStaticBusy;
      S     #FunctionStaticBusy;
      S     #FunctionBusy;
      R     #FunctionDone;
      L     0;
      T     #SFBError; // Systemfunktionsfehler werden zurueckgesetzt

NETWORK
TITLE =Datensatz Sollwert Leistung setzen

WRIT: NOP   0;
      CALL "AZYK_WR_SETVALUE" (
           START                    := TRUE,
           ID                       := DW#16#108,
           INDEX                    := 15,
           MAX_LAENGE               := 2,// Anzahl Bytes
           DBNUMMER                 := 159,// Datenbausteinnummer
           DATA_DONE                := #_SFBDone,
           SFB_BUSY                 := #_SFBBusy,
           SFB_ERROR                := #_SFBError,
           SFB_STATUS               := #_SFBStatus);

// Auswertung der Rueckgabewerte
      U     #_SFBBusy; // wenn die Funktion FC_AZYK_SETVALUE nicht beendet ist,
      SPB   ENDB; // dann Funktionsbaustein Ende
      U     #_SFBError; // wenn Funktion FC_AZYK_SETVALUE keinen Fehler meldet
      SPBN  RD_V; // dann LESEN VORBEREITEN
      SET   ; // Funktion FC_AZYK_SETVALUE hat einen Fehler gemeldet
      R     #FunctionBusy;
      R     #FunctionStaticBusy;
      R     #FunctionDPV1WriteDone;
      S     #FunctionDone;
      L     100; // S7 Fehlercode = 100 laden
      T     #SFBError; // Rueckgabe des Fehlercodes
      L     #_SFBStatus; // Funktionsbaustein Status laden
      T     #SFBStatusOut; // Rückgabe des S7 Fehlercodes
      BEA   ; // Funktionsbaustein wird abgebrochen
// Vorbereiten des DPV1 Lesedienst
RD_V: NOP   0;
      SET   ;
      S     #FunctionDPV1WriteDone; // nach erfolgreichem WRITEREC Flag setzen

NETWORK
TITLE =Datensatz Aktuelle Sollwerte auslesen

READ: NOP   0;
      CALL "AZYK_RD_DATABYTE" (
           START                    := TRUE,
           ID                       := DW#16#108,
           INDEX                    := 9,
           MAX_LAENGE               := 6,// Anzahl Bytes
           DBNUMMER                 := 154,// Datenbausteinnummer
           DATA_VALID               := #_SFBValid,
           SFB_BUSY                 := #_SFBBusy,
           SFB_ERROR                := #_SFBError,
           SFB_STATUS               := #_SFBStatus,
           LAENGE                   := #SFBRequestLength);

// Auswertung der Rueckgabewerte
      U     #_SFBBusy; // wenn die Funktion FC_AZYKRD_CURRSET nicht beendet ist,
      SPB   ENDB; // dann FunctionBusy Flag setzen
      U     #_SFBError; // wenn bei Datensatz schreiben kein Fehler aufgetreten ist
      SPBN  DATA; // dann Datenauswertung
      L     #TimeOutCounter;
      L     1;
      +I    ;
      T     #TimeOutCounter; // TimeOutCounter += 1
      L     #TimeOutCounter; // Wert von TimeOutCunter laden => AKKU1
      L     300; // Wert 300 laden => AKKU1 => TimeOutCounter => AKKU2
      >=I   ; // VKE = 1 bei AKKU2 >= AKKU1
      SPB   TOUT; // Springe bei VKE = 1 nach TOUT
// wenn der Fehler xx80B5xx gemeldet wird, dann liegt bereits ein anderer DPV1 Auftrag vor
      L     #_SFBStatus;
      UD    DW#16#FFFF00;
      L     DW#16#80B500;
      ==D   ;
// O
//L     #_SFCStatus
//UD    DW#16#FFFF00
//L     DW#16#80B200
//==D
      SPBN  ERR;
      NOP   0;
      SPA   ENDB;
// ein Fehler ist aufgetreten
ERR:  SET   ;
      R     #FunctionBusy;
      R     #FunctionStaticBusy;
      R     #FunctionDPV1WriteDone;
      S     #FunctionDone;
      L     100;
      T     #SFBError;
      L     #_SFBStatus;
      T     #SFBStatusOut;
      L     0;
      T     #TimeOutCounter; // Zeitzähler zurueck setzen
      BEA   ;
DATA: NOP   0;
      S     #FunctionDone;
      R     #FunctionBusy;
      R     #FunctionStaticBusy;
      R     #FunctionDPV1WriteDone;
      R     #FunctionActivate;
      L     0;
      T     #TimeOutCounter;
      BEA   ;

//Timeout
TOUT: NOP   0;
      L     2; // Fehlerwert 2
      T     #SFBError;
      L     0;
      T     #TimeOutCounter; // Zeitzaehler zurueck setzen
      SET   ;
      S     #FunctionDone;
      R     #FunctionActivate;
      R     #FunctionBusy;
      R     #_STATICBusy;
      R     #FunctionDPV1WriteDone;
      BEA   ;
NETWORK
TITLE =Funktionsbaustein definiert beenden

ENDB: SET   ;
      S     #FunctionBusy;
END:  NOP   0;

END_FUNCTION_BLOCK

DATA_BLOCK DB 126
TITLE =
VERSION : 0.0

"PS_AZYK_SETVAPOW_WRRD"
BEGIN
   SFBError := B#16#0;
   SFBStatusOut := DW#16#0;
   FunctionActivate := FALSE;
   FunctionBusy := FALSE;
   FunctionDone := FALSE;
   FunctionStaticBusy := FALSE;
   FunctionDPV1WriteDone := FALSE;
   TimeOutCounter := W#16#0;
   SFBRequestLength := 0;
   FunctionFlag := FALSE;
END_DATA_BLOCK

FUNCTION "CONVERT" : VOID
TITLE =
VERSION : 0.1

BEGIN
NETWORK
TITLE =

      AUF   "RDREC_DB_DEVNOMVALUE";



END_FUNCTION

FUNCTION "PARA_OVP_WR" : VOID
TITLE =PARAMETER SCHREIBEN
VERSION : 0.1


VAR_INPUT
  ADRESSE : INT ;
  DATEN : WORD ;
END_VAR
VAR_TEMP
  _ADRESSE : WORD ;
  _PAFE : INT ;
  _DATEN : WORD ;
END_VAR
BEGIN
NETWORK
TITLE =PARAMETER OVP SCHREIBEN
//Konsistentes Schreiben von Daten auf einen Slave (zyklisch)
      L     #ADRESSE;
      T     #_ADRESSE;

      L     #DATEN;
      T     #_DATEN;

      CALL "DPWR_DAT" (
           LADDR                    := #_ADRESSE,
           RECORD                   := #_DATEN,
           RET_VAL                  := #_PAFE);



END_FUNCTION

FUNCTION "PARA_WIDER_WR" : VOID
TITLE =PARAMETER KONSISTENT SCHREIBEN
VERSION : 0.1


VAR_INPUT
  ADRESSE : INT ;
  DATEN : WORD ;
END_VAR
VAR_TEMP
  _ADRESSE : WORD ;
  _PAFE : INT ;
  _DATEN : WORD ;
END_VAR
BEGIN
NETWORK
TITLE =PARAMETER WIDERSTAND SCHREIBEN

      L     #ADRESSE;
      T     #_ADRESSE;

      L     #DATEN;
      T     #_DATEN;

      CALL "DPWR_DAT" (
           LADDR                    := #_ADRESSE,
           RECORD                   := #_DATEN,
           RET_VAL                  := #_PAFE);

END_FUNCTION

FUNCTION "UniScale" : VOID
TITLE =Skalierfunktion allgemein
//Ein variabler Eingangsbereich wird auf einen variablen Ausgangsbereich
//skaliert. Eine Korrektur des Ausgangswertes in % ist möglich.
AUTHOR : IBNS
FAMILY : Mathe
NAME : UNIScale
VERSION : 0.1


VAR_INPUT
  Val : INT ;	//Eingangswert
  MinVal : INT ;	//Unterer Eingangsgrenzwert
  MaxVal : INT ;	//Oberer  Eingangsgrenzwert
  MinScal : INT ;	//Unterer skalierter Grenzwert
  MaxScal : INT ;	//Oberer  skalierter Grenzwert
  KorScal : INT ;	//Korrekturwert +/- in % für Ausgabewert
END_VAR
VAR_OUTPUT
  Scal : INT ;	//Skalierter Wert zwischen min/max
END_VAR
VAR_TEMP
  HubVal : INT ;	//Eingangshub
  HubScal : INT ;	//Ausgangshub
  TmpVal : INT ;	//Zwischenrgebniss
  Relation : REAL ;	//Relation Ausgangshub zu Eingangshub
  Korrektur : REAL ;	//Korrekturwert in %
END_VAR
BEGIN
NETWORK
TITLE =Scalierung durchführen

      L     #MaxVal;
      L     #MinVal;
      -I    ;
      T     #HubVal;

      L     #MaxScal;
      L     #MinScal;
      -I    ;
      T     #HubScal;

      L     #HubScal;
      ITD   ;
      DTR   ;
      L     #HubVal;
      ITD   ;
      DTR   ;
      /R    ;
      T     #Relation;

      L     #Val;
      L     #MinVal;
      -I    ;
      ITD   ;
      DTR   ;
      L     #Relation;
      *R    ;
      RND   ;
      L     #MinScal;
      +I    ;
      T     #TmpVal;

      L     #MinScal; // Ausgabebegrenzung auf min/max
      <I    ;
      SPB   NXT;
      TAK   ;
NXT:  L     #MaxScal;
      >I    ;
      SPB   out;
      TAK   ;
out:  T     #TmpVal;

NETWORK
TITLE =Korrekturwert berücksichtigen

      L     #KorScal;
      ITD   ;
      DTR   ;
      L     1.000000e+002;
      /R    ;
      L     1.000000e+000;
      +R    ;
      T     #Korrektur;
      L     #TmpVal;
      ITD   ;
      DTR   ;
      *R    ;
      RND   ;
      T     #Scal;

NETWORK
TITLE =Baustein Ende



END_FUNCTION

ORGANIZATION_BLOCK OB 1
TITLE = "Main Program Sweep (Cycle)"
VERSION : 0.1


VAR_TEMP
  OB1_EV_CLASS : BYTE ;	//Bits 0-3 = 1 (Coming event), Bits 4-7 = 1 (Event class 1)
  OB1_SCAN_1 : BYTE ;	//1 (Cold restart scan 1 of OB 1), 3 (Scan 2-n of OB 1)
  OB1_PRIORITY : BYTE ;	//Priority of OB Execution
  OB1_OB_NUMBR : BYTE ;	//1 (Organization block 1, OB1)
  OB1_RESERVED_1 : BYTE ;	//Reserved for system
  OB1_RESERVED_2 : BYTE ;	//Reserved for system
  OB1_PREV_CYCLE : INT ;	//Cycle time of previous OB1 scan (milliseconds)
  OB1_MIN_CYCLE : INT ;	//Minimum cycle time of OB1 (milliseconds)
  OB1_MAX_CYCLE : INT ;	//Maximum cycle time of OB1 (milliseconds)
  OB1_DATE_TIME : DATE_AND_TIME ;	//Date and time OB1 started
END_VAR
BEGIN
NETWORK
TITLE =Zyklischer Aufruf von FB10
//Zylkisches Lesen der Istwerte und des Gerätezustands
      UC    "PS_ZYKLISCH_DB10";

NETWORK
TITLE =Zyklischer Aufruf von FB11
//Zyklisches Schreiben der Sollwerte
      UC    "PS_ZYKL_SETVALUE";

NETWORK
TITLE =Datensatz Sollwert Spannung setzen / Aktuell(e) Sollwerte lesen
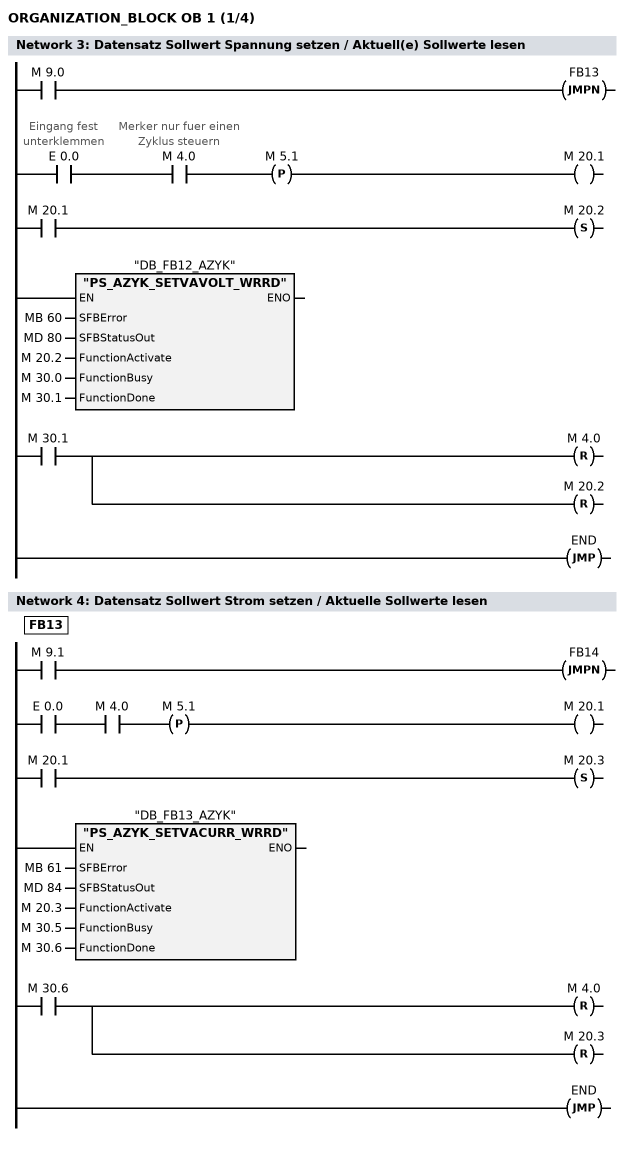
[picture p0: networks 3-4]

      U     M      9.0;
      SPBN  FB13;
      U     E      0.0; //Eingang fest unterklemmen
      U     M      4.0; //Merker nur fuer einen Zyklus steuern
      FP    M      5.1;
      =     M     20.1;

      U     M     20.1;
      S     M     20.2;

      CALL "PS_AZYK_SETVAVOLT_WRRD" , "DB_FB12_AZYK" (
           SFBError                 := MB    60,
           SFBStatusOut             := MD    80,
           FunctionActivate         := M     20.2,
           FunctionBusy             := M     30.0,
           FunctionDone             := M     30.1);

      U     M     30.1;
      R     M      4.0;
      R     M     20.2;
      SPA   END;

NETWORK
TITLE =Datensatz Sollwert Strom setzen / Aktuelle Sollwerte lesen

FB13: U     M      9.1;
      SPBN  FB14;
      U     E      0.0;
      U     M      4.0;
      FP    M      5.1;
      =     M     20.1;

      U     M     20.1;
      S     M     20.3;

      CALL "PS_AZYK_SETVACURR_WRRD" , "DB_FB13_AZYK" (
           SFBError                 := MB    61,
           SFBStatusOut             := MD    84,
           FunctionActivate         := M     20.3,
           FunctionBusy             := M     30.5,
           FunctionDone             := M     30.6);


      U     M     30.6;
      R     M      4.0;
      R     M     20.3;
      SPA   END;

NETWORK
TITLE =Datensatz Geraet Steuerung / Geraetemeldungen lesen
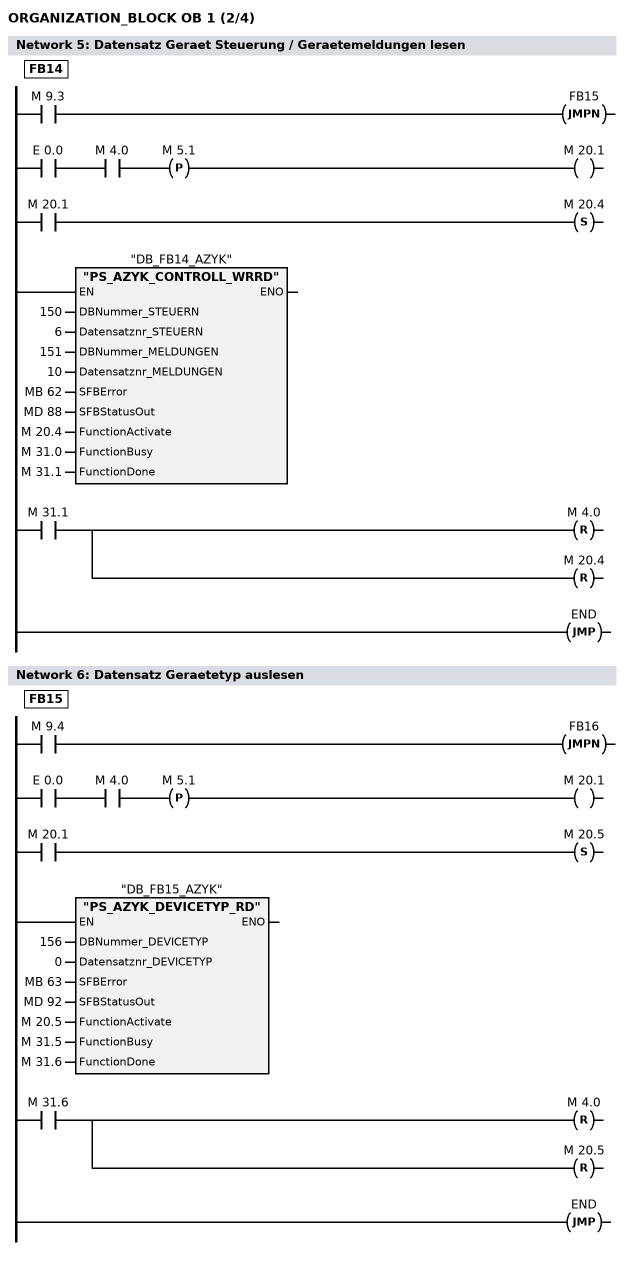
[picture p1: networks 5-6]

FB14: U     M      9.3;
      SPBN  FB15;
      U     E      0.0;
      U     M      4.0;
      FP    M      5.1;
      =     M     20.1;

      U     M     20.1;
      S     M     20.4;

      CALL "PS_AZYK_CONTROLL_WRRD" , "DB_FB14_AZYK" (
           DBNummer_STEUERN         := 150,
           Datensatznr_STEUERN      := 6,
           DBNummer_MELDUNGEN       := 151,
           Datensatznr_MELDUNGEN    := 10,
           SFBError                 := MB    62,
           SFBStatusOut             := MD    88,
           FunctionActivate         := M     20.4,
           FunctionBusy             := M     31.0,
           FunctionDone             := M     31.1);

      U     M     31.1;
      R     M      4.0;
      R     M     20.4;
      SPA   END;

NETWORK
TITLE =Datensatz Geraetetyp auslesen

FB15: U     M      9.4;
      SPBN  FB16;
      U     E      0.0;
      U     M      4.0;
      FP    M      5.1;
      =     M     20.1;

      U     M     20.1;
      S     M     20.5;

      CALL "PS_AZYK_DEVICETYP_RD" , "DB_FB15_AZYK" (
           DBNummer_DEVICETYP       := 156,
           Datensatznr_DEVICETYP    := 0,
           SFBError                 := MB    63,
           SFBStatusOut             := MD    92,
           FunctionActivate         := M     20.5,
           FunctionBusy             := M     31.5,
           FunctionDone             := M     31.6);

      U     M     31.6;
      R     M      4.0;
      R     M     20.5;
      SPA   END;
NETWORK
TITLE =Datensatz Geraeteartikelnummer auslesen
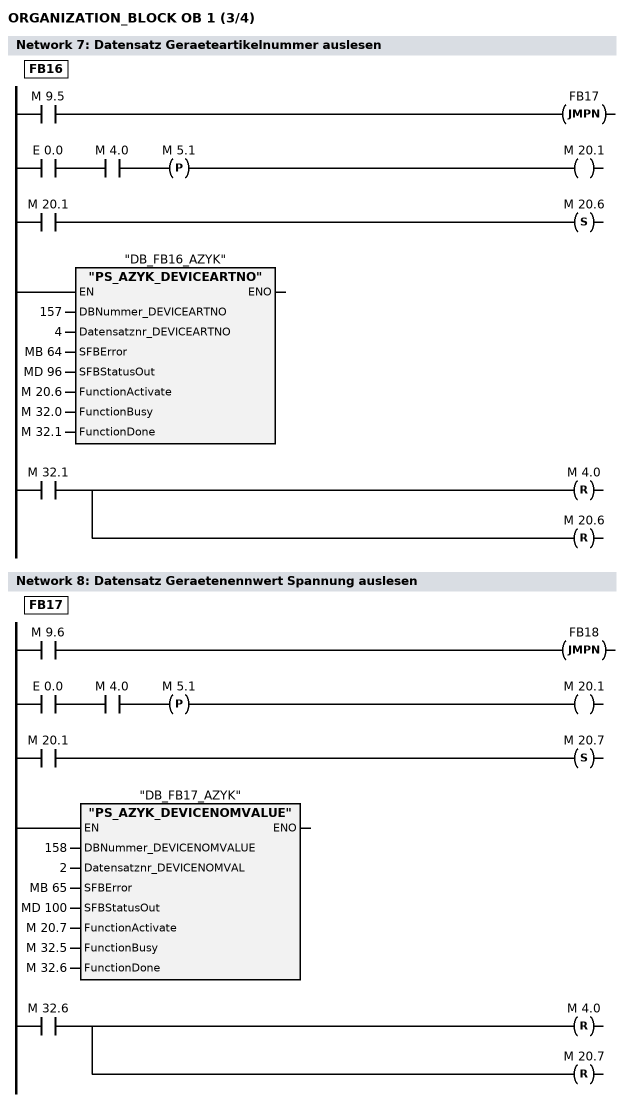
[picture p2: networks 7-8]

FB16: U     M      9.5;
      SPBN  FB17;
      U     E      0.0;
      U     M      4.0;
      FP    M      5.1;
      =     M     20.1;

      U     M     20.1;
      S     M     20.6;

      CALL "PS_AZYK_DEVICEARTNO" , "DB_FB16_AZYK" (
           DBNummer_DEVICEARTNO     := 157,
           Datensatznr_DEVICEARTNO  := 4,
           SFBError                 := MB    64,
           SFBStatusOut             := MD    96,
           FunctionActivate         := M     20.6,
           FunctionBusy             := M     32.0,
           FunctionDone             := M     32.1);

      U     M     32.1;
      R     M      4.0;
      R     M     20.6;
NETWORK
TITLE =Datensatz Geraetenennwert Spannung auslesen

FB17: U     M      9.6;
      SPBN  FB18;
      U     E      0.0;
      U     M      4.0;
      FP    M      5.1;
      =     M     20.1;

      U     M     20.1;
      S     M     20.7;

      CALL "PS_AZYK_DEVICENOMVALUE" , "DB_FB17_AZYK" (
           DBNummer_DEVICENOMVALUE  := 158,
           Datensatznr_DEVICENOMVAL := 2,
           SFBError                 := MB    65,
           SFBStatusOut             := MD   100,
           FunctionActivate         := M     20.7,
           FunctionBusy             := M     32.5,
           FunctionDone             := M     32.6);

      U     M     32.6;
      R     M      4.0;
      R     M     20.7;
NETWORK
TITLE =Datensatz Sollwert Leistung setzen / Aktuell(e) lesen
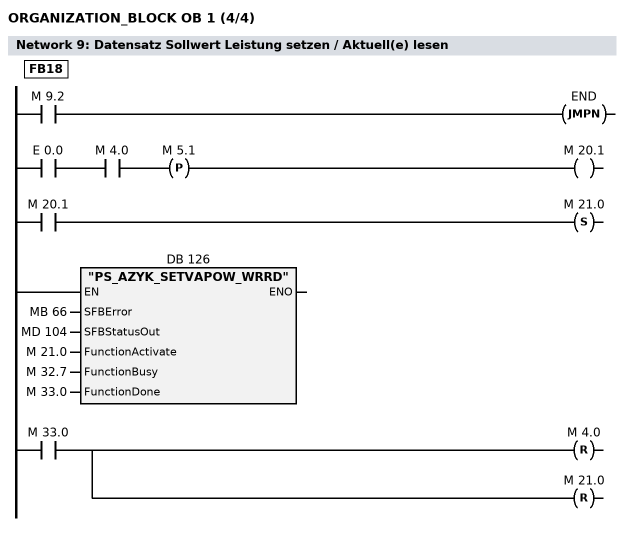
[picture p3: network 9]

FB18: U     M      9.2;
      SPBN  END;
      U     E      0.0;
      U     M      4.0;
      FP    M      5.1;
      =     M     20.1;

      U     M     20.1;
      S     M     21.0;

      CALL "PS_AZYK_SETVAPOW_WRRD" , DB   126 (
           SFBError                 := MB    66,
           SFBStatusOut             := MD   104,
           FunctionActivate         := M     21.0,
           FunctionBusy             := M     32.7,
           FunctionDone             := M     33.0);

      U     M     33.0;
      R     M      4.0;
      R     M     21.0;

NETWORK
TITLE =

END:  NOP   0;

NETWORK
TITLE =

      AUF   "PS_ZYK_DATEN";
      L     DBW    0;
      ITD   ; // Interger nach Double Interger
      DTR   ; // Double Interger nach Real
      T     MD   124;
      L     MD   124;


NETWORK
TITLE =Logisch 0 und Logisch 1

      O     M      1.0;
      ON    M      1.0;
      R     M      1.0;
      S     M      1.1;
END_ORGANIZATION_BLOCK

ORGANIZATION_BLOCK "DP: STATUS ALARM"
TITLE = "DP:status_alarm"
VERSION : 0.1


VAR_TEMP
  OB55_EV_CLASS : BYTE ;	//Bits 0-3 = 1 (Coming event), Bits 4-7 = 1 (Event class 1)
  OB55_STRT_INF : BYTE ;	//16#55 (OB 55 has started)
  OB55_PRIORITY : BYTE ;	//Priority of OB Execution
  OB55_OB_NUMBR : BYTE ;	//55 (Organization block 55, OB55)
  OB55_RESERVED_1 : BYTE ;	//Reserved for system
  OB55_IO_FLAG : BYTE ;	//16#54 (input module), 16#55 (output module)
  OB55_MDL_ADDR : WORD ;	//Base address of module initiating interrupt
  OB55_LEN : BYTE ;	//Length of information
  OB55_TYPE : BYTE ;	//Type of alarm
  OB55_SLOT : BYTE ;	//Slot
  OB55_SPEC : BYTE ;	//Specifier
  OB55_DATE_TIME : DATE_AND_TIME ;	//Date and time OB55 started
END_VAR
BEGIN
END_ORGANIZATION_BLOCK

ORGANIZATION_BLOCK "I/O_FLT1"
TITLE = "I/O Point Fault"
VERSION : 0.1


VAR_TEMP
  OB82_EV_CLASS : BYTE ;	//16#39, Event class 3, Entering event state, Internal fault event
  OB82_FLT_ID : BYTE ;	//16#XX, Fault identifcation code
  OB82_PRIORITY : BYTE ;	//Priority of OB Execution
  OB82_OB_NUMBR : BYTE ;	//82 (Organization block 82, OB82)
  OB82_RESERVED_1 : BYTE ;	//Reserved for system
  OB82_IO_FLAG : BYTE ;	//Input (01010100), Output (01010101)
  OB82_MDL_ADDR : WORD ;	//Base address of module with fault
  OB82_MDL_DEFECT : BOOL ;	//Module defective
  OB82_INT_FAULT : BOOL ;	//Internal fault
  OB82_EXT_FAULT : BOOL ;	//External fault
  OB82_PNT_INFO : BOOL ;	//Point information
  OB82_EXT_VOLTAGE : BOOL ;	//External voltage low
  OB82_FLD_CONNCTR : BOOL ;	//Field wiring connector missing
  OB82_NO_CONFIG : BOOL ;	//Module has no configuration data
  OB82_CONFIG_ERR : BOOL ;	//Module has configuration error
  OB82_MDL_TYPE : BYTE ;	//Type of module
  OB82_SUB_MDL_ERR : BOOL ;	//Sub-Module is missing or has error
  OB82_COMM_FAULT : BOOL ;	//Communication fault
  OB82_MDL_STOP : BOOL ;	//Module is stopped
  OB82_WTCH_DOG_FLT : BOOL ;	//Watch dog timer stopped module
  OB82_INT_PS_FLT : BOOL ;	//Internal power supply fault
  OB82_PRIM_BATT_FLT : BOOL ;	//Primary battery is in fault
  OB82_BCKUP_BATT_FLT : BOOL ;	//Backup battery is in fault
  OB82_RESERVED_2 : BOOL ;	//Reserved for system
  OB82_RACK_FLT : BOOL ;	//Rack fault, only for bus interface module
  OB82_PROC_FLT : BOOL ;	//Processor fault
  OB82_EPROM_FLT : BOOL ;	//EPROM fault
  OB82_RAM_FLT : BOOL ;	//RAM fault
  OB82_ADU_FLT : BOOL ;	//ADU fault
  OB82_FUSE_FLT : BOOL ;	//Fuse fault
  OB82_HW_INTR_FLT : BOOL ;	//Hardware interupt input in fault
  OB82_RESERVED_3 : BOOL ;	//Reserved for system
  OB82_DATE_TIME : DATE_AND_TIME ;	//Date and time OB82 started
END_VAR
BEGIN
END_ORGANIZATION_BLOCK

ORGANIZATION_BLOCK "OBNL_FLT"
TITLE = "Organization Block (OB) Not Loaded Fault"
VERSION : 0.1


VAR_TEMP
  OB85_EV_CLASS : BYTE ;	//16#35 Event class 3
  OB85_FLT_ID : BYTE ;	//16#XX, Fault identification code
  OB85_PRIORITY : BYTE ;	//Priority of OB Execution
  OB85_OB_NUMBR : BYTE ;	//85 (Organization block 85, OB85)
  OB85_RESERVED_1 : BYTE ;	//Reserved for system
  OB85_RESERVED_2 : BYTE ;	//Reserved for system
  OB85_RESERVED_3 : INT ;	//Reserved for system
  OB85_ERR_EV_CLASS : BYTE ;	//Class of event causing error
  OB85_ERR_EV_NUM : BYTE ;	//Number of event causing error
  OB85_OB_PRIOR : BYTE ;	//Priority of OB causing error
  OB85_OB_NUM : BYTE ;	//Number of OB causing error
  OB85_DATE_TIME : DATE_AND_TIME ;	//Date and time OB85 started
END_VAR
BEGIN
END_ORGANIZATION_BLOCK

ORGANIZATION_BLOCK "RACK_FLT"
TITLE = "Loss Of Rack Fault"
VERSION : 0.1


VAR_TEMP
  OB86_EV_CLASS : BYTE ;	//16#38/39 Event class 3
  OB86_FLT_ID : BYTE ;	//16#C1/C4/C5, Fault identifcation code
  OB86_PRIORITY : BYTE ;	//Priority of OB Execution
  OB86_OB_NUMBR : BYTE ;	//86 (Organization block 86, OB86)
  OB86_RESERVED_1 : BYTE ;	//Reserved for system
  OB86_RESERVED_2 : BYTE ;	//Reserved for system
  OB86_MDL_ADDR : WORD ;	//Base address of IM module in rack with fault
  OB86_RACKS_FLTD : ARRAY  [0 .. 31 ] OF BOOL ;	//Racks in fault
  OB86_DATE_TIME : DATE_AND_TIME ;	//Date and time OB86 started
  ERRORCode : INT ;
  REASON : INT ;
  ADDRESS : INT ;
  ERROR : BOOL ;
  FAILURE : BOOL ;
  RETURN : BOOL ;
END_VAR
BEGIN
NETWORK
TITLE =
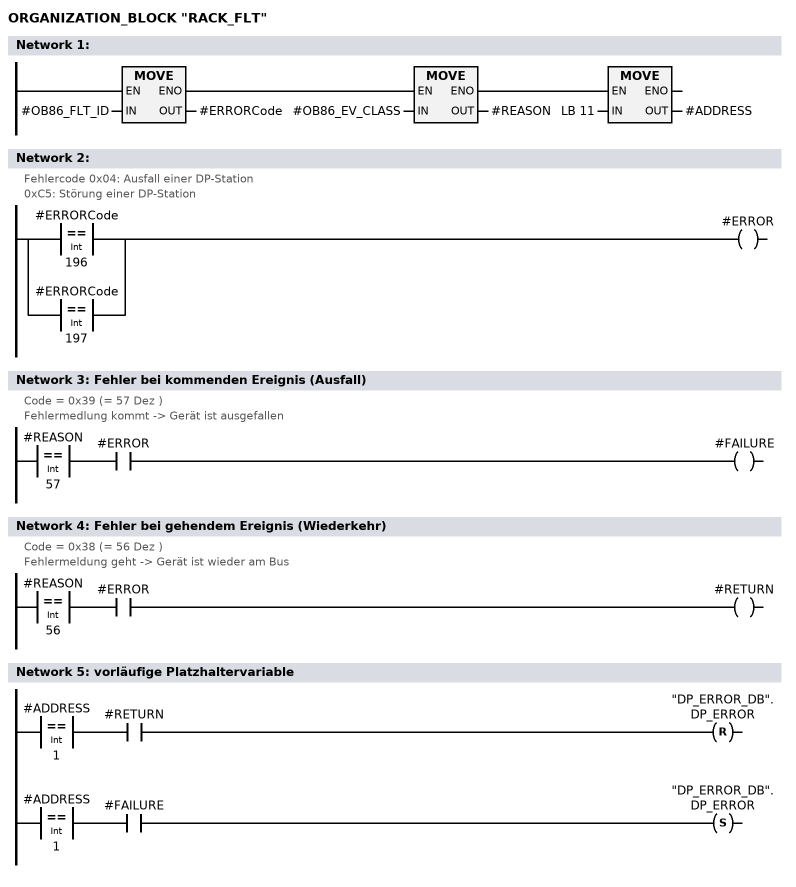
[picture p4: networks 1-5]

      L     #OB86_FLT_ID;
      T     #ERRORCode;

      L     #OB86_EV_CLASS;
      T     #REASON;

      L     LB    11;
      T     #ADDRESS;



NETWORK
TITLE =
//Fehlercode 0x04: Ausfall einer DP-Station
//           0xC5: Störung einer DP-Station


      O(    ;
      L     #ERRORCode;
      L     196;
      ==I   ;
      )     ;
      O(    ;
      L     #ERRORCode;
      L     197;
      ==I   ;
      )     ;
      =     #ERROR;
NETWORK
TITLE =Fehler bei kommenden Ereignis (Ausfall)
//Code = 0x39 (= 57 Dez )
//Fehlermedlung kommt -> Gerät ist ausgefallen
      U(    ;
      L     #REASON;
      L     57;
      ==I   ;
      )     ;
      U     #ERROR;
      =     #FAILURE;
NETWORK
TITLE =Fehler bei gehendem Ereignis (Wiederkehr)
//Code = 0x38 (= 56 Dez )
//Fehlermeldung geht -> Gerät ist wieder am Bus
      U(    ;
      L     #REASON;
      L     56;
      ==I   ;
      )     ;
      U     #ERROR;
      =     #RETURN;
NETWORK
TITLE =vorläufige Platzhaltervariable

      U(    ;
      L     #ADDRESS;
      L     1;
      ==I   ;
      )     ;
      U     #RETURN;
      R     "DP_ERROR_DB".DP_ERROR;
      U(    ;
      L     #ADDRESS;
      L     1;
      ==I   ;
      )     ;
      U     #FAILURE;
      S     "DP_ERROR_DB".DP_ERROR;
      NOP   0;
END_ORGANIZATION_BLOCK

ORGANIZATION_BLOCK "COMM_FLT"
TITLE = "Communication Fault"
VERSION : 0.1


VAR_TEMP
  OB87_EV_CLASS : BYTE ;	//16#39 Event class 3
  OB87_FLT_ID : BYTE ;	//16#XX, Fault identifcation code
  OB87_PRIORITY : BYTE ;	//Priority of OB Execution
  OB87_OB_NUMBR : BYTE ;	//87 (Organization block 87, OB87)
  OB87_RESERVED_1 : BYTE ;	//Reserved for system
  OB87_RESERVED_2 : BYTE ;	//Reserved for system
  OB87_RESERVED_3 : WORD ;	//Reserved for system
  OB87_RESERVED_4 : DWORD ;	//Reserved for system
  OB87_DATE_TIME : DATE_AND_TIME ;	//Date and time OB87 started
END_VAR
BEGIN
END_ORGANIZATION_BLOCK

ORGANIZATION_BLOCK "PROG_ERR"
TITLE = "Programming Error"
VERSION : 0.1


VAR_TEMP
  OB121_EV_CLASS : BYTE ;	//16#25, Event class 2, Entering event state, Internal fault event
  OB121_SW_FLT : BYTE ;	//16#XX Software programming fault
  OB121_PRIORITY : BYTE ;	//Priority of OB Execution
  OB121_OB_NUMBR : BYTE ;	//121 (Organization block 121, OB121)
  OB121_BLK_TYPE : BYTE ;	//16#88/8A/8B/8C/8E Type of block fault occured in
  OB121_RESERVED_1 : BYTE ;	//Reserved for system
  OB121_FLT_REG : WORD ;	//16#XX Specific register that caused fault
  OB121_BLK_NUM : WORD ;	//Number of block that programming fault occured in
  OB121_PRG_ADDR : WORD ;	//Address in block where programming fault occured
  OB121_DATE_TIME : DATE_AND_TIME ;	//Date and time OB121 started
END_VAR
BEGIN
END_ORGANIZATION_BLOCK

ORGANIZATION_BLOCK "MOD_ERR"
TITLE = "Module Access Error"
VERSION : 0.1


VAR_TEMP
  OB122_EV_CLASS : BYTE ;	//16#29, Event class 2, Entering event state, Internal fault event
  OB122_SW_FLT : BYTE ;	//16#XX Software error code
  OB122_PRIORITY : BYTE ;	//Priority of OB Execution
  OB122_OB_NUMBR : BYTE ;	//122 (Organization block 122, OB122)
  OB122_BLK_TYPE : BYTE ;	//16#88/8C/8E Type of block fault occured in
  OB122_MEM_AREA : BYTE ;	//Memory area where access error occured
  OB122_MEM_ADDR : WORD ;	//Memory address where access error occured
  OB122_BLK_NUM : WORD ;	//Block number in which error occured
  OB122_PRG_ADDR : WORD ;	//Program address where error occured
  OB122_DATE_TIME : DATE_AND_TIME ;	//Date and time OB1 started
END_VAR
BEGIN
END_ORGANIZATION_BLOCK

